FUNCTION "fc_h25_NoRunDG" : VOID
TITLE =Check, if no diesel running on the foreign busbars
//version!date    !author !change_segm!change_description
//-------+--------+-------+-----------+-------------------------------
// 1.0   !27.04.00!Kahle  ! ---       ! 1st version
// 1.1   !09.05.00!Kahle  ! 2,3       ! corr. program
AUTHOR : Kahle
FAMILY : PMA71_SC
NAME : NoFrgnDG
VERSION : 1.0


VAR_OUTPUT
  OUT_Noforeign_run : BOOL ;	//No diesel on the foreign busbars is running
  OUT_AtOneDG_run : BOOL ;	//At least one diesel is running on busbar
END_VAR
VAR_TEMP
  cfg_own : WORD ;	//configuration of the own busbar (of this shore connection)
  cfg_foreign : WORD ;	//configuration of the foreign busbars
  cfg_act : WORD ;	//actual configuration without shoreconnection, EG
  cnt_foreign : BYTE ;	//loop counter "foreign diesel"
  cnt_own : BYTE ;	//loop counter "own diesel"
  act_DB : WORD ;	//actual datablock ot the receive buffer
  foreignDG_run : BOOL ;	//at least one foreign diesel is running with closed generator breaker
  ownDG_run : BOOL ;	//at least one diesel is running on busbar
END_VAR
BEGIN
NETWORK
TITLE =Determine the configuration of the own busbar

      L     "prm_pma".p_bus_part;
      SLW   4; //convert to pointer *2 (=INT)
      LAR1  ;
      AUF   "prm_pma";
      L     DBW [AR1,P#22.0];
      L     W#16#1FFF;
      UW    ; //without EG, shore conn 1, shore conn 2
      T     #cfg_own; //configuration of the own busbar (of this shore connection)


NETWORK
TITLE =Determine the configuration of the foreign busbars

      L     "MEM".o51_actCfg;
      L     W#16#1FFF;
      UW    ; //configuration of the foreign busbar without EG, shore conn 1, shore conn 2
      L     #cfg_own;
      INVI  ;
      UW    ;
      T     #cfg_foreign;
NETWORK
TITLE =Check if a diesel is running on the foreign busbars

      CLR   ;
      =     #foreignDG_run;
      L     13;
lpfg: T     #cnt_foreign;
      L     #cfg_foreign;
      SRW   ;
      SPZ   nxfg; //no diesel defined ...next one

      L     #cnt_foreign;
      +     108;
      T     #act_DB;

      AUF   DB [#act_DB];
      UN    DBX   38.2; //f_brk_clseG1
      SPB   nxfg; //breaker not closed ...next one

      S     #foreignDG_run; //breaker closed -->set flag

nxfg: L     #cnt_foreign;
      LOOP  lpfg;

NETWORK
TITLE =output parameter

      UN    #foreignDG_run;
      =     #OUT_Noforeign_run;

NETWORK
TITLE =Determine the configuration of the own busbars or common busbar

      L     "MEM".o51_actCfg;
      L     W#16#1FFF;
      UW    ; //configuration of the own busbar without EG, shore conn 1, shore conn 2
      T     #cfg_act;
NETWORK
TITLE =Check if a diesel is running on the own busbars

      CLR   ;
      =     #ownDG_run;
      L     13;
lpow: T     #cnt_own;
      L     #cfg_act;
      SRW   ;
      SPZ   nxow; //no diesel defined ...next one

      L     #cnt_own;
      +     108;
      T     #act_DB;

      AUF   DB [#act_DB];
      UN    DBX   38.2; //f_brk_clseG1
      SPB   nxow; //breaker not closed ...next one

      S     #ownDG_run; //breaker closed -->set flag

nxow: L     #cnt_own;
      LOOP  lpow;

      U     #ownDG_run;
      =     #OUT_AtOneDG_run;
END_FUNCTION


FUNCTION "fc_h22_TotLoad" : VOID
TITLE =calculation of the total power of the actual busbar
AUTHOR : Kahle
FAMILY : PMA71
NAME : MeanValu
VERSION : 1.0


VAR_INPUT
  IN_actCfg : WORD ;	//actual configuration (.0:G1 - .12:G13, .13/.14:S1,S2 , .15:EG)
END_VAR
VAR_OUTPUT
  OUT_total_load : DINT ;	//Total load [kW]
  OUT_No_busbar : INT ;	//Number of generator on busbar
END_VAR
VAR_TEMP
  MPI_cnt : BYTE ;	//MPI received data area loop counter
  MPI_DB : INT ;	//MPI received DB
  load_total : DINT ;	//temporary total load [kW]
  Onbus_No : BYTE ;	//Number of generators on busbar
END_VAR
BEGIN
NETWORK
TITLE =intial.internal variables

      L     0;
      T     #load_total;
      T     #Onbus_No;
NETWORK
TITLE =calculate the mean value of the load signals

      L     14;
lpmv: T     #MPI_cnt;
      L     #IN_actCfg;
      SRW   ;
      SPZ   nxmv; //if generator'x' no defined then ...next one

      L     #MPI_cnt;
      +     108;
      T     #MPI_DB;
      AUF   DB [#MPI_DB];

// check if generator'x' on bus
      U     DBX   38.2;
      SPBN  onbs; //if f_brk_clse' =false then ...next one

//add up the actual load
      L     DBW   42;
      ITD   ;
      L     #load_total;
      +D    ;
      T     #load_total; //a_loadG'x'

//add number of generators on busbar
onbs: U     DBX   38.3;
      SPBN  nxmv; //if f_onbus =false then ...next one
      L     #Onbus_No;
      +     1;
      T     #Onbus_No;

//next generator
nxmv: L     #MPI_cnt;

      LOOP  lpmv;

//output
      L     #load_total;
      T     #OUT_total_load;
      L     #Onbus_No;
      T     #OUT_No_busbar;
END_FUNCTION

FUNCTION_BLOCK "fb_522_addAlarm"
TITLE =Additional shore connection protection function (->FB56)
AUTHOR : Kahle
FAMILY : PMA71_SC
NAME : SC_Alarm
VERSION : 1.0


VAR_INPUT
  in_PrtcEG_sign : DWORD ;	//Protection signals especially emergency diesel
END_VAR
VAR_OUTPUT
  out_Fail_Warn_Curr_I : BOOL ;	//Indication "warning Overcurrent I"
  out_Fail_Warn_Curr_II : BOOL ;	//Indication "warning Overcurrent II"
  out_Fail_Warn_Load_I : BOOL ;	//Indication "warning Load I"
  out_Fail_Warn_Load_II : BOOL ;	//Indication "warning Load II"
END_VAR
VAR_TEMP
  temp_Limit_I1 : BOOL ;	//Generator current, limit 1 exceeded (Standby start)
  temp_Limit_I2 : BOOL ;	//Generator current, limit 2 exceeded (Standby start)
  temp_Limit_I3 : BOOL ;	//Generator current, limit 3 exceeded (Uness. consumers 1)
  temp_Limit_I4 : BOOL ;	//Generator current, limit 4 exceeded (Uness. consumers 2)
  temp_Limit_I5 : BOOL ;	//Generator current, limit 5 exceeded (Uness. consumers 3)
  temp_Limit_I6 : BOOL ;	//Generator current, limit 6 exceeded (Standby start, Uness. consumers 1-3)
  temp_Limit_I7 : BOOL ;	//Generator current, limit 7 exceeded (Generator breaker Off)
  temp_Limit_P1 : BOOL ;	//Generator load, limit 1 exceeded (Standby start)
  temp_Limit_P2 : BOOL ;	//Generator load, limit 2 exceeded (Standby start)
  temp_Limit_P3 : BOOL ;	//Generator load, limit 3 exceeded (Uness. consumers 1)
  temp_Limit_P4 : BOOL ;	//Generator load, limit 4 exceeded (Uness. consumers 2)
  temp_Limit_P5 : BOOL ;	//Generator load, limit 5 exceeded (Uness. consumers 3)
  temp_Limit_P6 : BOOL ;	//Generator load, limit 6 exceeded (Standby start, Uness. consumers 1, 2, 3)
  temp_Limit_P7 : BOOL ;	//Generator load, limit 7 exceeded (Gen. breaker Off)
  temp_Limit_f1 : BOOL ;	//Busbar frequency, limit 1 exceeded (Standby start)
  temp_Limit_f2 : BOOL ;	//Busbar frequency, limit 2 exceeded (Standby start)
  temp_Limit_f3 : BOOL ;	//Busbar frequency, limit 3 exceeded (Uness. consumers 1)
  temp_Limit_f4 : BOOL ;	//Busbar frequency, limit 4 exceeded (Uness. consumers 2)
  temp_Limit_f5 : BOOL ;	//Busbar frequency, limit 5 exceeded (Uness. consumers 3)
  temp_Limit_f6 : BOOL ;	//Busbar frequency, limit 6 exceeded (Standby start, Uness. consumers 1, 2, 3)
  temp_Limit_f7 : BOOL ;	//Busbar frequency, limit 7 exceeded (Gen. breaker Off)
  temp_Limit_f8 : BOOL ;	//Busbar frequency, limit 8 exceeded (Overfrequency alarm)
  temp_Limit_U1 : BOOL ;	//Busbar voltage, limit 1 exceeded (Undervoltage, standby start)
  temp_Limit_U2 : BOOL ;	//Busbar voltage, limit 2 exceeded (Undervoltage, Gen. breaker Off)
  temp_Limit_U3 : BOOL ;	//Busbar voltage, limit 3 exceeded (Overvoltage, standby start)
  temp_Limit_U4 : BOOL ;	//Busbar voltage, limit 4 exceeded (Overvoltage, blocking of voltage controller)
  temp_Limit_P7_undel : BOOL ;	//Generator load, limit 7 exceeded, undelayed (Gen. breaker Off)
  temp_Limit_P7_Warn : BOOL ;	//Generator load, limit 7 exceeded, protection warning
  temp_ShortCircuit : BOOL ;	//Latch for signal "Short circuit"
  temp_Wind_Overtemp : BOOL ;	//Generator winding overtemperature, time delayed
  temp_Standby_ProtWarn : BOOL ;	//Request for standby start (EG: Protection warning)
  temp_Uness1_TransfLBrk : BOOL ;	//Trip command for unessential consumers 1 (EG: Trip of transfer line CB)
  temp_Harb_Feedb_Mode : BOOL ;	//Emergency generator in harbour mode or in power feedback mode
END_VAR
BEGIN
NETWORK
TITLE =Load protection signals into the internal store
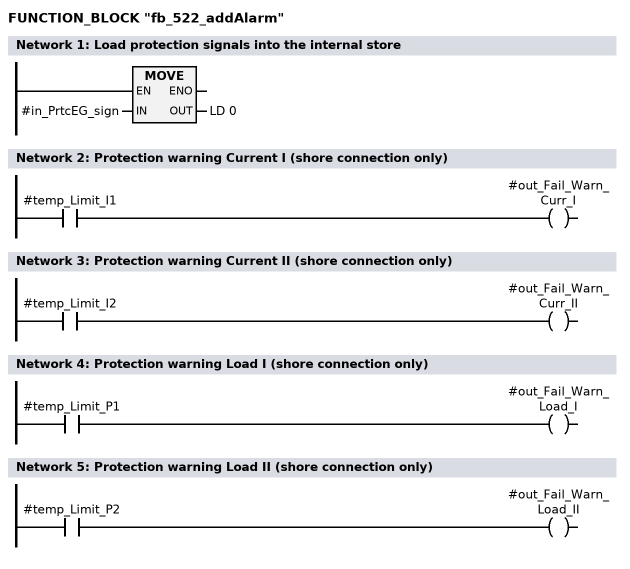
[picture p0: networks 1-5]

      L     #in_PrtcEG_sign;
      T     LD     0; //temp_Limit_I1...
NETWORK
TITLE =Protection warning Current I (shore connection only)

      U     #temp_Limit_I1;
      =     #out_Fail_Warn_Curr_I;
NETWORK
TITLE =Protection warning Current II (shore connection only)

      U     #temp_Limit_I2;
      =     #out_Fail_Warn_Curr_II;
NETWORK
TITLE =Protection warning Load I (shore connection only)

      U     #temp_Limit_P1;
      =     #out_Fail_Warn_Load_I;
NETWORK
TITLE =Protection warning Load II (shore connection only)

      U     #temp_Limit_P2;
      =     #out_Fail_Warn_Load_II;
END_FUNCTION_BLOCK

FUNCTION_BLOCK "fc_522_adjustVolt"
TITLE =Adjusting voltage busbar/ shore connection
//version!date    !author !change_segm!change_description
//-------+--------+-------+-----------+-------------------------------
// 1.0   !01.03.00!Kahle  ! ---       ! 1st version
// 1.1   !18.04.00!Kahle  ! 1(new)    !store signal "adjusting active"
//       !        !       ! 2,3       !signal "#stat_adjustActive" instead of
//       !        !       !           !       "IN_req_adjust"
//       !        !       ! 3         !signal "OUT_adjust" independent from signal
//       !        !       !           !       "#OUT_voltOK_mem
//  1.2  !19.04.00!Kahle  ! 1         !start timer "adjusting voltage"
//       !        !       ! 2         !limit "voltage difference" adjustable
//       !        !       ! 3         !conditions for output "OUT_adjust" are
//       !        !       !           !changed
//  1.3  !09.05.00!Kahle  ! div       !new para: start monit.T
//       !        !       !           !
//       !        !       !           !
//       !        !       !           !
//       !        !       !           !
//       !        !       !           !
//       !        !       !           !
//
AUTHOR : Kahle
FAMILY : PMA71
NAME : AjstVolt
VERSION : 1.3


VAR_INPUT
  IN_strt_adjust : BOOL ;	//start adjusting voltage between busbar and shore connection
  IN_stp_adjust : BOOL ;	//stop adjusting voltage between busbar and shore connection
  IN_strt_wait : BOOL ;	//start waiting time "adjusting voltage"
  IN_bus_L1_L2 : INT ;	//voltage busbar L1/L2
  IN_bus_L3_L1 : INT ;	//voltage busbar L3/L1
  IN_bus_L2_L3 : INT ;	//voltage busbar L2/L3
  IN_shore_L1_L2 : INT ;	//voltage shore connection L1/L2
  IN_shore_L3_L1 : INT ;	//voltage shore connection L3/L1
  IN_shore_L2_L3 : INT ;	//voltage shore connection L2/L3
  IN_Timer_dlyTAdjust : TIMER ;	//Timer "delay time voltage adjusting"
  IN_Timer_MonitAdjust : TIMER ;	//Timer "monitoring voltage adjusting"
  IN_reset : BOOL ;	//Reset failure
END_VAR
VAR_OUTPUT
  OUT_adjust : BOOL ;	//Adjusting voltage
  OUT_failAdjust : BOOL ;	//Failure: Adjusting voltage
END_VAR
VAR_IN_OUT
  OUT_voltOK_mem : BOOL ;	//Voltage between busbar and shore connection ok
END_VAR
VAR
  stat_adjustActive : BOOL ;	//Voltage adjusting is active
  stat_waitTAdjust : BOOL ;	//Waiting time "adjusting" is active
  stat_adjustFail : BOOL ;	//Failure: adjusting voltage
END_VAR
VAR_TEMP
  temp_L1L2unequal : BOOL ;	//voltage L1_L2 between busbar and shore connection is not equal
  temp_L1L3unequal : BOOL ;	//voltage L1_L3 between busbar and shore connection is not equal
  temp_L2L3unequal : BOOL ;	//voltage L2_L3 between busbar and shore connection is not equal
  temp_L1L2equal : BOOL ;	//voltage L1_L2 between busbar and shore connection is equal
  temp_L1L3equal : BOOL ;	//voltage L1_L3 between busbar and shore connection is equal
  temp_L2L3equal : BOOL ;	//voltage L2_L3 between busbar and shore connection is equal
END_VAR
BEGIN
NETWORK
TITLE =Store "voltage adjusting"
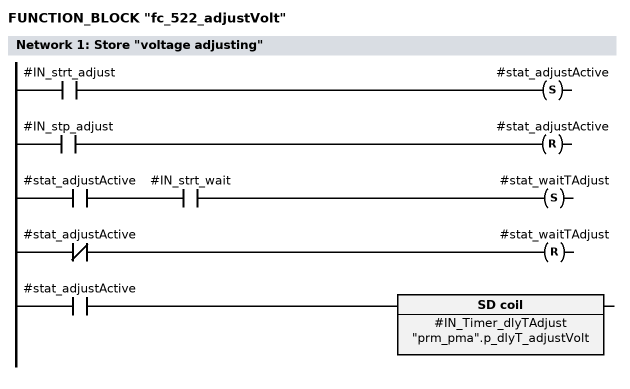
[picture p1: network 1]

      U     #IN_strt_adjust;
      S     #stat_adjustActive;
      U     #IN_stp_adjust;
      R     #stat_adjustActive;

      U     #stat_adjustActive;
      U     #IN_strt_wait;
      S     #stat_waitTAdjust;
      UN    #stat_adjustActive;
      R     #stat_waitTAdjust;

      U     #stat_adjustActive;
      L     "prm_pma".p_dlyT_adjustVolt;
      SE    #IN_Timer_dlyTAdjust;

NETWORK
TITLE =Check voltage between busbar and shore connection and each phas

      UN    #stat_adjustActive;
      SPB   time;

//Check voltage between busbar and shore connection and each phases
      L     #IN_bus_L1_L2;
      L     #IN_shore_L1_L2;
      -I    ;
      PUSH  ;
      SRD   16;
      POP   ;
      SPZ   pos1; //if difference positive ...jump
      NEGI  ;
pos1: L     "I_prtcSR".s_U_DIFF_SET;
      <I    ;
      =     #temp_L1L2equal;
      TAK   ;
      L     "prm_pma".p_allowVoltDiff; //U_DIFF_SET - delta(V)
      -I    ;
      L     "I_prtcSR".s_U_DIFF_SET;
      >I    ;
      =     #temp_L1L2unequal;

      L     #IN_bus_L3_L1;
      L     #IN_shore_L3_L1;
      -I    ;
      PUSH  ;
      SRD   16;
      POP   ;
      SPZ   pos3; //if difference positive ...jump
      NEGI  ;
pos3: L     "I_prtcSR".s_U_DIFF_SET;
      <I    ;
      =     #temp_L1L3equal;
      TAK   ;
      L     "prm_pma".p_allowVoltDiff; //U_DIFF_SET - delta(V)
      -I    ;
      L     "I_prtcSR".s_U_DIFF_SET;
      >I    ;
      =     #temp_L1L3unequal;

      L     #IN_bus_L2_L3;
      L     #IN_shore_L2_L3;
      -I    ;
      PUSH  ;
      SRD   16;
      POP   ;
      SPZ   pos2; //if difference positive ...jump
      NEGI  ;
pos2: L     "I_prtcSR".s_U_DIFF_SET;
      <I    ;
      =     #temp_L2L3equal;
      TAK   ;
      L     "prm_pma".p_allowVoltDiff; //U_DIFF_SET - delta(V)
      -I    ;
      L     "I_prtcSR".s_U_DIFF_SET;
      >I    ;
      =     #temp_L2L3unequal;

      U     #temp_L1L2equal;
      U     #temp_L1L3equal;
      U     #temp_L2L3equal;
      S     #OUT_voltOK_mem;

      O     #temp_L1L2unequal;
      O     #temp_L1L3unequal;
      O     #temp_L2L3unequal;
      R     #OUT_voltOK_mem;


NETWORK
TITLE =Adjusting the voltage between busbar and shore connection
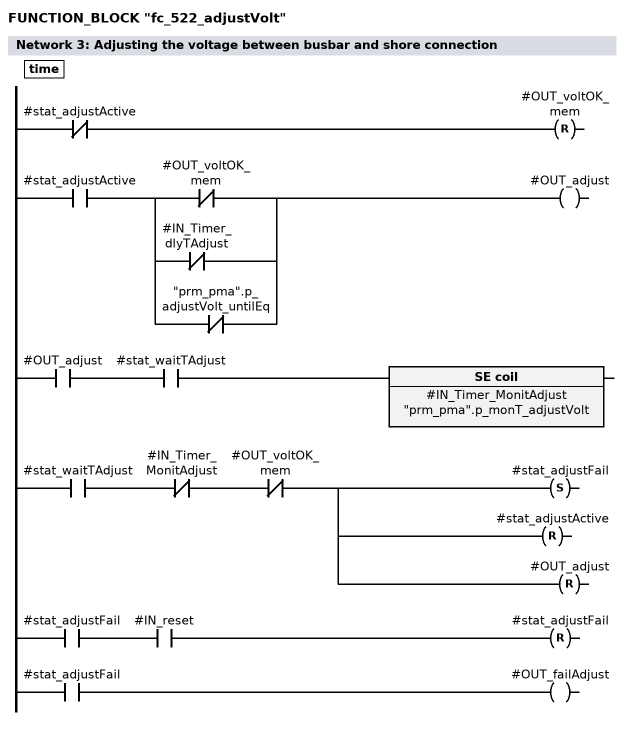
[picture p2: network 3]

time: ON    #stat_adjustActive;
      R     #OUT_voltOK_mem;

      U     #stat_adjustActive;
      U(    ;
      ON    #OUT_voltOK_mem;
      ON    #IN_Timer_dlyTAdjust;
      ON    "prm_pma".p_adjustVolt_untilEq;
      )     ;
      =     #OUT_adjust;

//monitoring time for adjusting voltage
      U     #OUT_adjust;
      U     #stat_waitTAdjust;
      L     "prm_pma".p_monT_adjustVolt;
      SV    #IN_Timer_MonitAdjust;

//monitoring time finished without compensation
      U     #stat_waitTAdjust;
      UN    #IN_Timer_MonitAdjust;
      UN    #OUT_voltOK_mem;
      S     #stat_adjustFail;
      R     #stat_adjustActive;
      R     #OUT_adjust;

      U     #stat_adjustFail;
      U     #IN_reset;
      R     #stat_adjustFail;

      U     #stat_adjustFail;
      =     #OUT_failAdjust;
END_FUNCTION_BLOCK

FUNCTION_BLOCK "fb_522_shoreConn"
TITLE =Shore connection monitoring
//This program controlled the following functions:
//
// - Check the release conditions
// - Lock / release the controller in the generator sets
// - Monitoring of the shutdown criteria
//
//version!date    !author !change_segm!change_description
//-------+--------+-------+-----------+-------------------------------
// 1.0   !26.03.00!Kahle  ! ---       ! 1st version
// 1.1   !18.04.00!Kahle  ! 30        ! Call FB82, new parameter "stop_adjusting"
//       !        !       ! 37        ! add.signal at the para. "IN_simLock"
// 1.2   !09.05.00!Kahle  ! 30        ! parameter "stop_adjusting": shore conn.on
//       !        !       ! 37(new)   ! Adjust voltage whether shore disconn.
//       !        !       ! 37(new    ! Indication "disconn. shore connection"
//       !        !       ! 27        ! signal "shore voltage" connected with
//       !        !       !           ! selector "im-/export"
//       !        !       ! 19(new)   ! Ind "blackout out shore connection"
//       !        !       ! 28        ! external release: new signal "shore on"
//       !        !       !           !                 : "voltage busbar" conn.
//       !        !       !           !                 : with selector
//       !        !       ! 27,28     ! external release: no diesel running on
//       !        !       !           !                   the foreign busbars
//       !        !       ! 42        ! blackout -signal
//       !        !       ! 19,20(new)! blackout monitoring busbar
//       !        !       ! 4,5(new)  ! change selector
//       !        !       ! 26        ! add.alarm "standby start"
//       !        !       ! 29(new)   ! common signal "blackout"
//       !        !       ! 35        ! Start/stop volt.adjust:new commands
//       !        !       ! 36        ! Stop Diesel: signals are changed
//       !        !       ! 38        ! Warn.Stop DG: signals are changed
//       !        !       ! 39        ! Open breaker: signals are changed
//       !        !       ! 40(new)   ! Alarm "DG doesn't stop"
//       !        !       ! 41(new)   ! Signal "absolute value of load signal"
//       !        !       ! 44        ! add signal "selector"
//       !        !       ! 45        ! reset "#stat_indShore_dis" add.signals
//       !        !       ! 46        ! stop adjust.: add.signals
//       !        !       ! 47(new)   ! Alarm "standby start failure"
//       !        !       ! 48        ! reset "#step1_c_brk_off": add.signals
//       !        !       ! 49        ! Alarm "take over load"
//       !        !       ! 50        ! Var.changes "Failure Diesel takeover load"
//       !        !       ! 51        ! Var.changes "Diesel takeover load(import)
//       !        !       ! 52(new)   ! Diesel take over load (mode =export)
//       !        !       ! 53(new)   ! Diesel take over load INDICATION
//       !        !       ! 54        ! Parameter "GB open with red": add.signal
//       !        !       !           ! Parameter "PB GB open": new signal
//       !        !       ! 58        ! Alarm "standby" deleted
//       !        !       ! 59(new)   ! Alarm "standby"
//       !        !       ! 60(new)   ! Alarm "blackout expected"
//       !        !       ! 77        ! Add.signals "blocked"
// 1.3   !20.07.00!Kahle  ! 26,59     ! Alarm'standbyStart" external few sec.only
// 1.4   !14.05.01!Kahle  ! 23        ! Add.ind "OUT_e_I_ov" & "OUT_e_P_ov"
//       !        !       ! 54        ! Add.signals "IN_extShoreBrk_openCmd",
//       !        !       !           ! Add.signals "IN_extBlock"
//
AUTHOR : Kahle
FAMILY : PMA71_SC
NAME : TieMonit
VERSION : 1.4


VAR_INPUT
  IN_selector : BOOL ;	//=0: IMPORT, =1: EXPORT
  IN_cmd_ShoreBrk_on : BOOL ;	//Command shore breaker on
  IN_cmd_ShoreBrk_off : BOOL ;	//Command shore breaker off
  IN_PB_ShoreBrk_off : BOOL ;	//PB shore conn breaker off
  IN_extShoreBrk_openCmd : BOOL ;	//External shore connection open command
  IN_extBlock : BOOL ;	//External blocking is active
  IN_blackout_bus : BOOL ;	//Blackout is detected on the busbar
  IN_VoltAvail_bus : BOOL ;	//Voltage available on the busbar
  IN_blackout_shore : BOOL ;	//Blackout is detected on the shore connection
  IN_shoreVoltAvail : BOOL ;	//Voltage on the shore connection is available
  IN_shortCircuit_otherG : BOOL ;	//At least one generator set has a short circuit detected
  IN_atLeastOneAuto : BOOL ;	//At least one generator set is in automatic
  IN_shortCircuit_ext : BOOL ;	//External device has a short circuit dedected
  IN_atLeastOneAutoOnbus : BOOL ;	//At least one generator set on bus in automatic
  IN_atLeastOneBrkClse : BOOL ;	//At least one generator set is on the busbar
  IN_atLeastShoreOn : BOOL ;	//At least one shore connection is on
  IN_atLeastDGrun : BOOL ;	//At least ond generator set is running
  IN_actCfg : WORD ;	//Actual configuration
  IN_GEN_I_L1 : INT ;	//GENOP71: I_L1
  IN_GEN_I_L2 : INT ;	//GENOP71: I_L2
  IN_GEN_I_L3 : INT ;	//GENOP71: I_L3
  IN_LOAD : INT ;	//GENOP71: active power [in kW]
  IN_BUS_f : INT ;	//GENOP71: f_bus
  IN_GEN_f : INT ;	//GENOP71: f_gen
  IN_BUS_U_L1L2 : INT ;	//GENOP71: U_L1L2_bus
  IN_BUS_U_L2L3 : INT ;	//GENOP71: U_L2L3_bus
  IN_BUS_U_L1L3 : INT ;	//GENOP71: U_L1L3_bus
  IN_GEN_U_L1L2 : INT ;	//GENOP71: U_L1L2_gen
  IN_GEN_U_L2L3 : INT ;	//GENOP71: U_L2L3_gen
  IN_GEN_U_L1L3 : INT ;	//GENOP71: U_L1L3_gen
  IN_I_SC_GW1 : BOOL ;	//GENOP71: I_SC_GW1
  IN_I_GW1VER : BOOL ;	//GENOP71: I_GW1VER
  IN_I_GW2VER : BOOL ;	//GENOP71: I_GW2VER
  IN_I_GW3VER : BOOL ;	//GENOP71: I_GW3VER
  IN_I_GW4VER : BOOL ;	//GENOP71: I_GW4VER
  IN_P_GW1VER : BOOL ;	//GENOP71: P_GW1VER
  IN_simLock_blc : BOOL ;	//Simultaneous lock is blocked
  IN_simLock_err : BOOL ;	//Simultaneous lock failure
  IN_simLockRel : BOOL ;	//Simultaneous lock release
  IN_shoreBrk_trip : BOOL ;	//Shore breaker tripped
  IN_brk_ready : BOOL ;	//Breaker is ready for closing
  IN_brk_normPos : BOOL ;	//Breaker is in norm position
  IN_brk_testPos : BOOL ;	//Breaker is in test position
  IN_brk_on : BOOL ;	//Feedback: breaker is on
  IN_brk_off : BOOL ;	//Feedback: breaker is off
  IN_f_cmdBrkOn : BOOL ;	//Genop Feedback: command breaker on
  IN_reset : BOOL ;	//Reset command
  IN_resetBlock : BOOL ;	//Reset blocking
  IN_pressCnfrm : BOOL ;	//indication: press confirmation
  IN_mode : BYTE ;	//Actual mode (x.0:local, x.1:semiOP, x.2:autoOP, x.3:semi, x.4:auto, x.5:test)
  IN_TimerStdbyStrt : TIMER ;	//Timer startpulse "standby start"
  IN_TimerStpGenSet : TIMER ;	//Timer monitoring generator set stop
  IN_TimerStpPulse : TIMER ;	//Timer stoppulse "diesel"
  IN_TimerMonStdbyStrt : TIMER ;	//Timer monitoring generator set start
  IN_TimerTakeLoad : TIMER ;	//Timer monitoring take over load generator set
END_VAR
VAR_OUTPUT
  OUT_SynchrActive : BOOL ;	//Command: switch up/down
  OUT_c_LckCtrl : BOOL ;	//Command: controller lock
  OUT_c_simLock : BOOL ;	//Command: simultanoeus lock active
  OUT_c_brkON : BOOL ;	//GENOP Command: breaker on
  OUT_c_brkOFF : BOOL ;	//GENOP Command: breaker off
  OUT_c_synRel : BOOL ;	//GENOP Command: synchronizing release
  OUT_c_reqStrt : BOOL ;	//Command: request standby start
  OUT_c_reqStp : BOOL ;	//Command: request stop generator set
  OUT_c_adjustVolt : BOOL ;	//Command: Adjusting voltage
  OUT_c_takeoverLoad : BOOL ;	//Command: take over load
  OUT_c_shortCirc : BOOL ;	//Command: short circuit, open breaker
  OUT_i_blocked : BOOL ;	//Indication: shore connection is blocked
  OUT_i_disconn : BOOL ;	//Indication: disconning shore connection
  OUT_stdbyNo_1st : BYTE ;	//Number of the actual standby generator
  OUT_e_busbar_monit : BOOL ;	//Failure: busbar monitoring
  OUT_e_shore_monit : BOOL ;	//Failure: shore connection monitoring
  OUT_e_I_monit : BOOL ;	//Failure: current monitoring
  OUT_e_I : BOOL ;	//Failure: CB tripped by overcurrent
  OUT_e_revP : BOOL ;	//Failure: reverse power (active in "export" mode)
  OUT_e_I_ov : BOOL ;	//Failure: overcurrent 1
  OUT_e_P_ov : BOOL ;	//Failure: overload 1
  OUT_e_f1 : BOOL ;	//Failure: underfrequency 1
  OUT_e_f2 : BOOL ;	//Failure: underfrequency 2
  OUT_e_f3 : BOOL ;	//Failure: underfrequency 3
  OUT_e_f4 : BOOL ;	//Failure: overfrequency
  OUT_e_U1 : BOOL ;	//Failure: undervoltage 1
  OUT_e_U2 : BOOL ;	//Failure: undervoltage 2
  OUT_e_U3 : BOOL ;	//Failure: undervoltage 3
  OUT_e_U4 : BOOL ;	//Failure: overvoltage
  OUT_e_I_sc : BOOL ;	//Failure: short circuit
  OUT_e_sc_other : BOOL ;	//Failure: short circuit at other generator set
  OUT_e_I1 : BOOL ;	//Failure: overcurrent I
  OUT_e_I2 : BOOL ;	//Failure: overcurrent II
  OUT_e_P1 : BOOL ;	//Failure: overload I
  OUT_e_P2 : BOOL ;	//Failure: overload II
  OUT_e_black : BOOL ;	//Failure: blackout
  OUT_e_brkRdy : BOOL ;	//Failure: breaker ready
  OUT_e_brkOn : BOOL ;	//Failure: breaker on
  OUT_e_brkOff : BOOL ;	//Failure: breaker off
  OUT_e_brkOnOff : BOOL ;	//Failure: breaker feedbak plausibility
  OUT_e_brkTrip : BOOL ;	//Failure: breaker tripped
  OUT_e_brkTripExt : BOOL ;	//Failure: shore connection breaker tripped extern
  OUT_e_synTime : BOOL ;	//Failure: synchronization time exceeded
  OUT_e_StdbyStart : BOOL ;	//Failure: standby start
  OUT_e_loadTooHigh : BOOL ;	//Failure: Power consumption is too high
  OUT_e_adjustVolt : BOOL ;	//Failure: Adjusting voltage
  OUT_e_warnBlackout : BOOL ;	//Warning: Danger of blackout because of no generator set in automatic
  OUT_e_alarmBlackout : BOOL ;	//Alarm: Danger of blackout because of no generator set in automatic
  OUT_e_stpDieselMan : BOOL ;	//Alarm: Stop diesel manually in case of starting shore connection
  OUT_e_noStpDiesel : BOOL ;	//Alarm: No shore conn in case of no DG stop
  OUT_e_standByStart : BOOL ;	//Alarm: Start standby diesel
  OUT_e_takeOverLoad : BOOL ;	//Alarm: Take over load
  OUT_w_takeOverLoad : BOOL ;	//Warning: Take over load manually
  OUT_ind_ready : BYTE ;	//indication: criteria for breaker ready
  OUT_ind_line1_stat : INT ;	//status indication -line 1-
  out_ind_line2_var : INT ;	//status indication -line 2-
END_VAR
VAR
  Gen_Protect : "fb_511_GenProtect";
  Gen_Breaker : "fb_57_clseopnBrk";
  Add_Warning : "fb_522_addAlarm";
  BlockShoreCnn : BOOL ;	//Shore connection breaker is blocked
  BothSideBlackout : BOOL ;	//Blackout on the entire busbar
  BrkRdyClse : BOOL ;	//Breaker is ready for closing
  Pulse_brk_on : BOOL ;	//Pulse "breaker on"
  step1_c_brk_off : BOOL ;	//Command store "breaker off" -step 1-
  step2_c_brk_off : BOOL ;	//Command store "breaker off" -step 2-
  stat_relSimLock : BOOL ;	//Release simultaneous lock after voltage adjusting
  stat_relClseGenBrk : BOOL ;	//Release close generator breaker
  stat_indShore_dis : BOOL ;	//Disconnecting shore connection is active
  stat_c_shore_on : BOOL ;	//Memory command shore connection on
  stat_negP_TimerStpDG : BOOL ;	//Negative pulse timer "stop diesel"
  stat_failStandBy : BOOL ;	//Failure start standby diesel
  stat_failTakeOver : BOOL ;	//Failure take over load
  stat_failBlackout_SC : BOOL ;	//Failure Blackout shore connection
  stat_selector_imp : BOOL ;	//Memo selector =import
  stat_selector_exp : BOOL ;	//Memo selector =export
  Breaker_control : "fb_57_clseopnBrk";	//Breaker control (close, open, monitoring)
  AdjustVolt_conn : "fc_522_adjustVolt";	//Adjusting voltage whether the shore connection will be connected
  AdjustVolt_disconn : "fc_522_adjustVolt";	//Adjusting voltage whether the shore connection will be disconnected
END_VAR
VAR_TEMP
  temp_OM_Local : BOOL ;	//Active operation mode: Local
  temp_OM_Semi_OP : BOOL ;	//Active operation mode: Semi automatic OP
  temp_OM_Auto_OP : BOOL ;	//Active operation mode: Automatic OP
  temp_OM_Semi_MMI : BOOL ;	//Active operation mode: Semi automatic MMI
  temp_OM_Auto_MMI : BOOL ;	//Active operation mode: Automatic MMI
  temp_OM_Test : BOOL ;	//Active operation mode: Test (EG only)
  temp_Reserve_006 : BOOL ;	//Reserved (Transfer Byte --> Bit)
  temp_Reserve_007 : BOOL ;	//Reserved (Transfer Byte --> Bit)
  temp_ext_release : BOOL ;	//external releases
  temp_shoreBus_on : BOOL ;	//shore connection active at the configuration 1
  temp_shoreTrs_on : BOOL ;	//shore connection active at the configuration 2
  temp_TieOffBlack : BOOL ;	//On side blackout: tie breaker off
  temp_TieOffNoGen : BOOL ;	//Number of allowed generator exceeded: tie breaker off
  temp_req_StdbyStrt : BOOL ;	//Request start standby generator set
  temp_VoltAvailBusPrtct : BOOL ;	//Busbar voltage available
  temp_VoltAvailShorePrtct : BOOL ;	//Shore connection voltage available
  temp_Brk_off : BOOL ;	//Command: breaker off
  temp_block : BOOL ;	//Blocking own breaker
  temp_Auto : BOOL ;	//mode =automatic OP or automatic MMI
  temp_c_brkOff : BOOL ;	//command: breaker off
  temp_c_brkLoadRed : BOOL ;	//command: shore connection breaker off with load reduction
  temp_tieBrk_ready : BOOL ;	//tie breaker ready
  var26 : BOOL ;
  var27 : BOOL ;
  temp_VoltAvailBus : BOOL ;	//voltage busbar available
  temp_VoltAvailShore : BOOL ;	//voltage shore connection available
  temp_blocking : BOOL ;	//Shore connection is blocked
  temp_LoadTooHigh : BOOL ;	//Total load is too high
  temp_Semi : BOOL ;	//Active operation mode: Semi automatic
  temp_normTestPos : BOOL ;	//Breaker in norm or test position
  temp_readyClose : BOOL ;	//Breaker is ready for closing
  temp_brkOff_noLoad : BOOL ;	//Breaker off, load less then minimum
  temp_GEN_I_L1 : INT ;	//Generator current L1 (in 100.00% of nominal value)
  temp_GEN_I_L2 : INT ;	//Generator current L1 (in 100.00% of nominal value)
  temp_GEN_I_L3 : INT ;	//Generator current L1 (in 100.00% of nominal value)
  temp_BUS_f : INT ;	//Bus bar frequency (in 100.00% of nominal value)
  temp_GEN_f : INT ;	//Generator frequency (in 100.00% of nominal value)
  temp_BUS_U_L1L2 : INT ;	//Bus bar voltage L1/L2 (in 100.00% of nominal value)
  temp_BUS_U_L2L3 : INT ;	//Bus bar voltage L2/L3 (in 100.00% of nominal value)
  temp_GEN_P_SUM : INT ;	//Generator active load (in 100.00% of nominal value)
  temp_Operat_Status : INT ;	//status indication for OP7
  temp_BUS_U_L3L1 : INT ;	//Bus bar voltage L3/L1 (in 100.00% of nominal value)
  temp_GEN_U_L1L2 : INT ;	//Generator voltage L1/L2 (in 100.00% of nominal value)
  temp_GEN_U_L2L3 : INT ;	//Generator voltage L2/L3 (in 100.00% of nominal value)
  temp_GEN_U_L3L1 : INT ;	//Generator voltage L3/L1 (in 100.00% of nominal value)
  temp_GenNo_onbus : INT ;	//Number of generator which are on busbar
  temp_CfgBusbar : INT ;	//Actual configration busbar
  temp_CfgTrans : INT ;	//Actual configuration transferline
  temp_Indication2_FB51 : INT ;	//Indication number, line 2, from FB51
  temp_totalLoad : DINT ;	//total load of the actual configuration
  temp_No_busbar : INT ;	//Number of generator in automatic on busbar
  temp_addAlarm : DWORD ;	//Additional shore connection warnings
  temp_c_adjustV_conn : BOOL ;	//command "adjusting voltage" in case connecting to shore
  temp_c_adjustV_disconn : BOOL ;	//command "adjusting voltage" in case disconnecting from shore
  temp_e_adjustV_conn : BOOL ;	//failure "adjusting voltage" in case connecting to shore
  temp_e_adjustV_disconn : BOOL ;	//failure "adjusting voltage" in case disconnecting from shore
  temp_e_blackout : BOOL ;	//failure "blackout shore connection"
  temp_noForeignRun : BOOL ;	//No running diesel on foreign busbars
  temp_atOneDG_run : BOOL ;	//At least one diesel is running on busbar
  temp_blackBus : BOOL ;	//blackout on the busbar
  temp_e_alarmBlack_I : BOOL ;	//Alarm: Blackout expected
  temp_e_alarmBlack_II : BOOL ;	//Alarm: Blackout expected
  temp_blackout : BOOL ;	//blackout
  temp_e_standby_ext : BOOL ;	//Alarm: standby start external
  temp_e_standby_int : BOOL ;	//Alarm: standby start internal
  temp_selec_chgToExp : BOOL ;	//Selector change to export
  temp_selec_chgToImp : BOOL ;	//Selector change to import
  temp_reset_actProcess : BOOL ;	//Reset actual process
  temp_open_withoutRed : BOOL ;	//Open shore connection without load reduction
  temp_GEN_U_Max : INT ;	//Mains (generator) voltage, highest value (phase L1/L2, L2/L3, L3/L1)
END_VAR
BEGIN
NETWORK
TITLE =GENERAL -Move operation mode (Transfer Byte --> Bit)
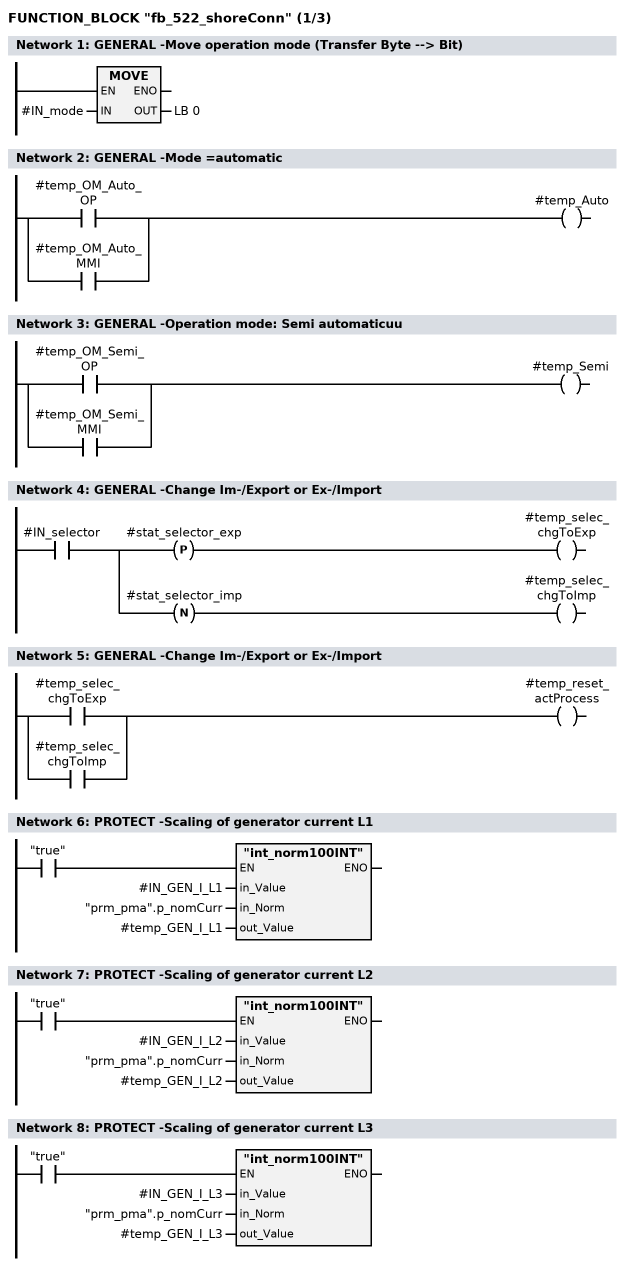
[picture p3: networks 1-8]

      L     #IN_mode;
      T     LB     0;
NETWORK
TITLE =GENERAL -Mode =automatic

      O     #temp_OM_Auto_OP;
      O     #temp_OM_Auto_MMI;
      =     #temp_Auto;
NETWORK
TITLE =GENERAL -Operation mode: Semi automaticuu

      O     #temp_OM_Semi_OP;
      O     #temp_OM_Semi_MMI;
      =     #temp_Semi;
NETWORK
TITLE =GENERAL -Change Im-/Export or Ex-/Import

      U     #IN_selector;
      =     L     54.0;
      U     L     54.0;
      FP    #stat_selector_exp;
      =     #temp_selec_chgToExp;
      U     L     54.0;
      FN    #stat_selector_imp;
      =     #temp_selec_chgToImp;
NETWORK
TITLE =GENERAL -Change Im-/Export or Ex-/Import

      O     #temp_selec_chgToExp;
      O     #temp_selec_chgToImp;
      =     #temp_reset_actProcess;
NETWORK
TITLE =PROTECT -Scaling of generator current L1

      U     "true";
      SPBNB _001;
      CALL "int_norm100INT" (
           in_Value                 := #IN_GEN_I_L1,
           in_Norm                  := "prm_pma".p_nomCurr,
           out_Value                := #temp_GEN_I_L1);
_001: NOP   0;
NETWORK
TITLE =PROTECT -Scaling of generator current L2

      U     "true";
      SPBNB _002;
      CALL "int_norm100INT" (
           in_Value                 := #IN_GEN_I_L2,
           in_Norm                  := "prm_pma".p_nomCurr,
           out_Value                := #temp_GEN_I_L2);
_002: NOP   0;
NETWORK
TITLE =PROTECT -Scaling of generator current L3

      U     "true";
      SPBNB _003;
      CALL "int_norm100INT" (
           in_Value                 := #IN_GEN_I_L3,
           in_Norm                  := "prm_pma".p_nomCurr,
           out_Value                := #temp_GEN_I_L3);
_003: NOP   0;
NETWORK
TITLE =PROTECT -Scaling of busbar frequency
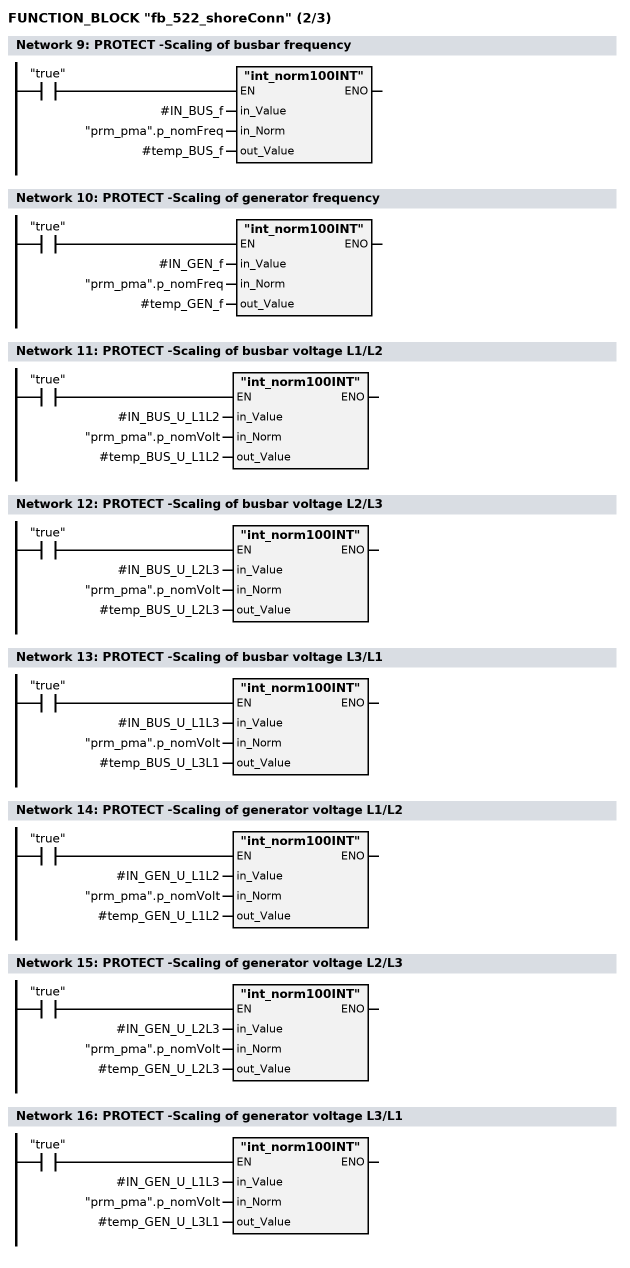
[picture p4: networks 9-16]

      U     "true";
      SPBNB _007;
      CALL "int_norm100INT" (
           in_Value                 := #IN_BUS_f,
           in_Norm                  := "prm_pma".p_nomFreq,
           out_Value                := #temp_BUS_f);
_007: NOP   0;
NETWORK
TITLE =PROTECT -Scaling of generator frequency

      U     "true";
      SPBNB _00b;
      CALL "int_norm100INT" (
           in_Value                 := #IN_GEN_f,
           in_Norm                  := "prm_pma".p_nomFreq,
           out_Value                := #temp_GEN_f);
_00b: NOP   0;
NETWORK
TITLE =PROTECT -Scaling of busbar voltage L1/L2

      U     "true";
      SPBNB _011;
      CALL "int_norm100INT" (
           in_Value                 := #IN_BUS_U_L1L2,
           in_Norm                  := "prm_pma".p_nomVolt,
           out_Value                := #temp_BUS_U_L1L2);
_011: NOP   0;
NETWORK
TITLE =PROTECT -Scaling of busbar voltage L2/L3

      U     "true";
      SPBNB _012;
      CALL "int_norm100INT" (
           in_Value                 := #IN_BUS_U_L2L3,
           in_Norm                  := "prm_pma".p_nomVolt,
           out_Value                := #temp_BUS_U_L2L3);
_012: NOP   0;
NETWORK
TITLE =PROTECT -Scaling of busbar voltage L3/L1

      U     "true";
      SPBNB _013;
      CALL "int_norm100INT" (
           in_Value                 := #IN_BUS_U_L1L3,
           in_Norm                  := "prm_pma".p_nomVolt,
           out_Value                := #temp_BUS_U_L3L1);
_013: NOP   0;
NETWORK
TITLE =PROTECT -Scaling of generator voltage L1/L2

      U     "true";
      SPBNB _017;
      CALL "int_norm100INT" (
           in_Value                 := #IN_GEN_U_L1L2,
           in_Norm                  := "prm_pma".p_nomVolt,
           out_Value                := #temp_GEN_U_L1L2);
_017: NOP   0;
NETWORK
TITLE =PROTECT -Scaling of generator voltage L2/L3

      U     "true";
      SPBNB _01b;
      CALL "int_norm100INT" (
           in_Value                 := #IN_GEN_U_L2L3,
           in_Norm                  := "prm_pma".p_nomVolt,
           out_Value                := #temp_GEN_U_L2L3);
_01b: NOP   0;
NETWORK
TITLE =PROTECT -Scaling of generator voltage L3/L1

      U     "true";
      SPBNB _01c;
      CALL "int_norm100INT" (
           in_Value                 := #IN_GEN_U_L1L3,
           in_Norm                  := "prm_pma".p_nomVolt,
           out_Value                := #temp_GEN_U_L3L1);
_01c: NOP   0;
NETWORK
TITLE =PROTECT -Scaling of generator active load
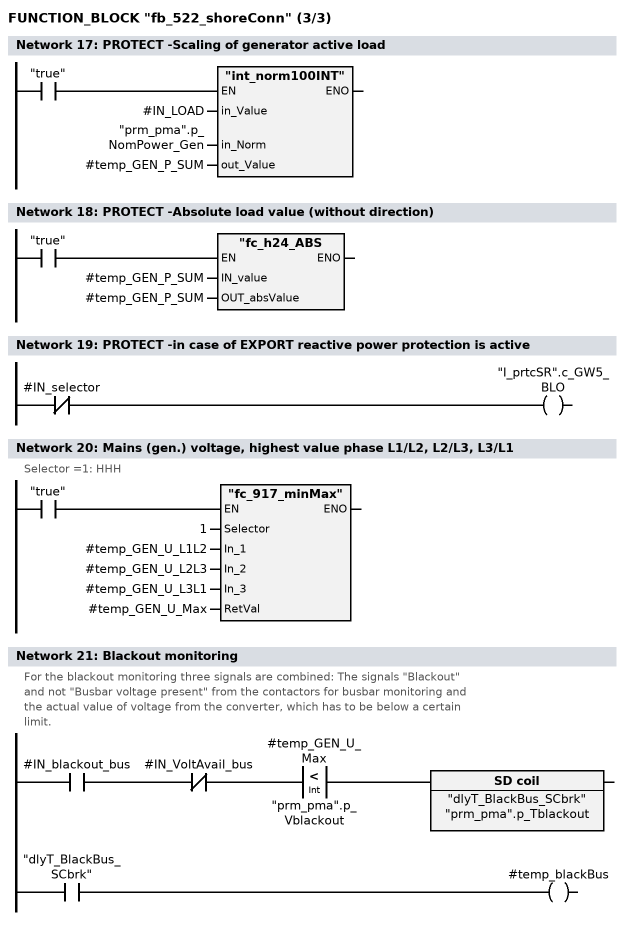
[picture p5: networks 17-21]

      U     "true";
      SPBNB _01d;
      CALL "int_norm100INT" (
           in_Value                 := #IN_LOAD,
           in_Norm                  := "prm_pma".p_NomPower_Gen,
           out_Value                := #temp_GEN_P_SUM);
_01d: NOP   0;
NETWORK
TITLE =PROTECT -Absolute load value (without direction)

      U     "true";
      SPBNB _01e;
      CALL "fc_h24_ABS(INT)" (
           IN_value                 := #temp_GEN_P_SUM,
           OUT_absValue             := #temp_GEN_P_SUM);
_01e: NOP   0;
NETWORK
TITLE =PROTECT -in case of EXPORT reactive power protection is active

      UN    #IN_selector;
      =     "I_prtcSR".c_GW5_BLO;
NETWORK
TITLE =Mains (gen.) voltage, highest value phase L1/L2, L2/L3, L3/L1
//Selector =1: HHH
      U     "true";
      SPBNB _01f;
      CALL "fc_917_minMax" (
           Selector                 := 1,
           In_1                     := #temp_GEN_U_L1L2,
           In_2                     := #temp_GEN_U_L2L3,
           In_3                     := #temp_GEN_U_L3L1,
           RetVal                   := #temp_GEN_U_Max);
_01f: NOP   0;
NETWORK
TITLE =Blackout monitoring
//For the blackout monitoring three signals are combined: The signals "Blackout"
//and not "Busbar voltage present" from the contactors for busbar monitoring and
//the actual value of voltage from the converter, which has to be below a certain
//limit.
      U     #IN_blackout_bus;
      UN    #IN_VoltAvail_bus;
      U(    ;
      L     #temp_GEN_U_Max;
      L     "prm_pma".p_Vblackout;
      <I    ;
      )     ;
      L     "prm_pma".p_Tblackout;
      SE    "dlyT_BlackBus_SCbrk";
      NOP   0;
      NOP   0;
      NOP   0;
      U     "dlyT_BlackBus_SCbrk";
      =     #temp_blackBus;
NETWORK
TITLE =Indication "Failure busbar/blackout monitoring"
//If both signals "Blackout" and "Busbar voltage present" from the contactors for
//busbar monitoring are present or both are not present, there is a failure in
//the
//busbar monitoring.
      U     #IN_reset;
      R     #OUT_e_busbar_monit;
      U(    ;
      U(    ;
      U     #IN_blackout_bus;
      U     #IN_VoltAvail_bus;
      O     ;
      UN    #IN_blackout_bus;
      UN    #IN_VoltAvail_bus;
      )     ;
      L     "prm_pma".p_TFBusbar;
      SE    "dlyT_BusbarFail_SCbrk";
      NOP   0;
      NOP   0;
      NOP   0;
      U     "dlyT_BusbarFail_SCbrk";
      )     ;
      S     #OUT_e_busbar_monit;
      NOP   0;
NETWORK
TITLE =PROTECT -Generator protection (FB56)
//In this case: Generator means busbar, busbar means transferline!
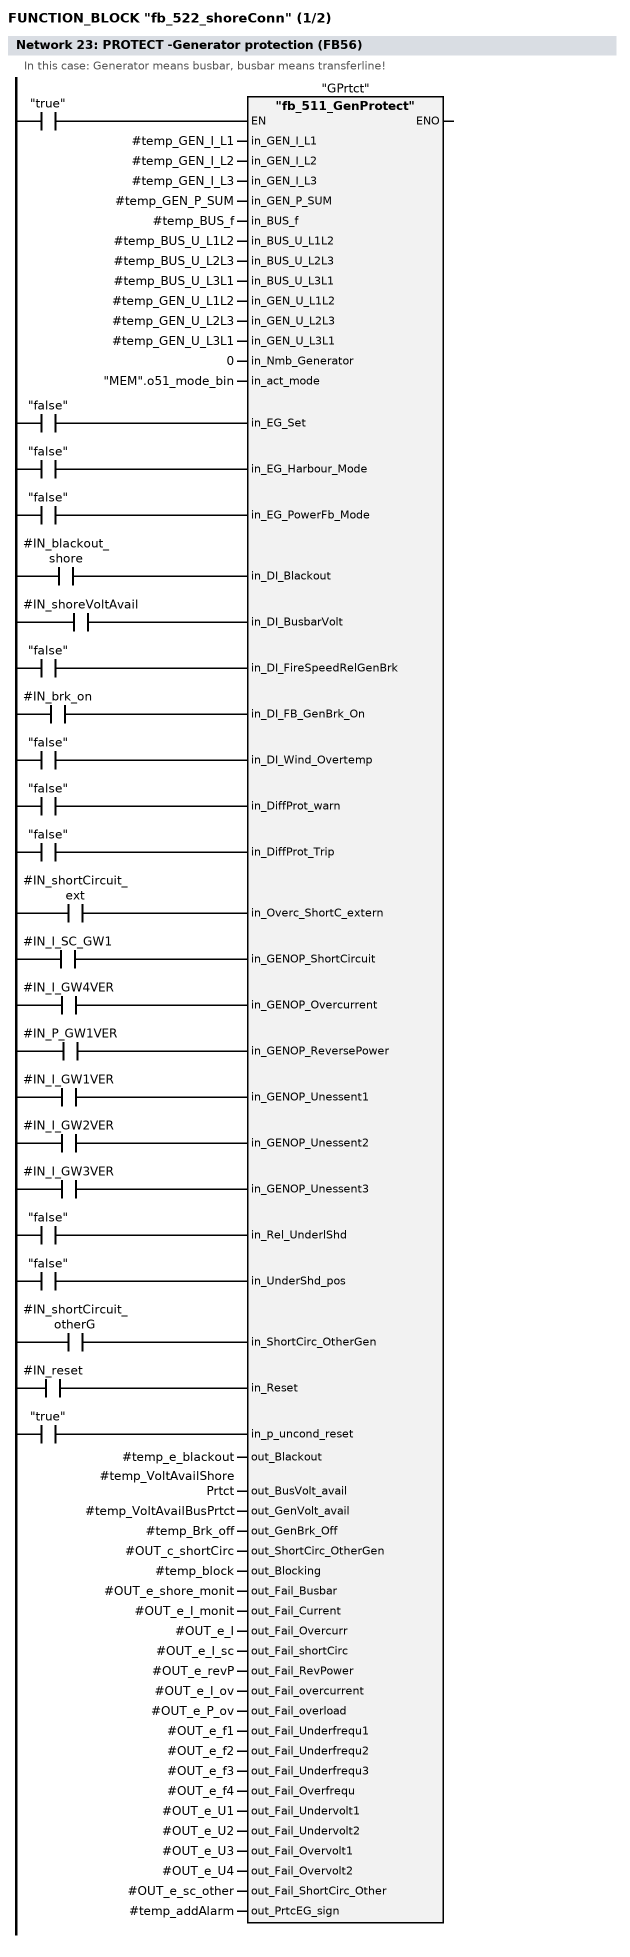
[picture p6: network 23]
      U     "false";
      =     L     54.0;
      BLD   103;
      U     "false";
      =     L     54.1;
      BLD   103;
      U     "false";
      =     L     54.2;
      BLD   103;
      U     #IN_blackout_shore;
      =     L     54.3;
      BLD   103;
      U     #IN_shoreVoltAvail;
      =     L     54.4;
      BLD   103;
      U     "false";
      =     L     54.5;
      BLD   103;
      U     #IN_brk_on;
      =     L     54.6;
      BLD   103;
      U     "false";
      =     L     54.7;
      BLD   103;
      U     "false";
      =     L     55.0;
      BLD   103;
      U     "false";
      =     L     55.1;
      BLD   103;
      U     #IN_shortCircuit_ext;
      =     L     55.2;
      BLD   103;
      U     #IN_I_SC_GW1;
      =     L     55.3;
      BLD   103;
      U     #IN_I_GW4VER;
      =     L     55.4;
      BLD   103;
      U     #IN_P_GW1VER;
      =     L     55.5;
      BLD   103;
      U     #IN_I_GW1VER;
      =     L     55.6;
      BLD   103;
      U     #IN_I_GW2VER;
      =     L     55.7;
      BLD   103;
      U     #IN_I_GW3VER;
      =     L     56.0;
      BLD   103;
      U     "false";
      =     L     56.1;
      BLD   103;
      U     "false";
      =     L     56.2;
      BLD   103;
      U     #IN_shortCircuit_otherG;
      =     L     56.3;
      BLD   103;
      U     #IN_reset;
      =     L     56.4;
      BLD   103;
      U     "true";
      =     L     56.5;
      BLD   103;
      U     "true";
      SPBNB _024;
      CALL "fb_511_GenProtect" , "GPrtct" (
           in_GEN_I_L1              := #temp_GEN_I_L1,
           in_GEN_I_L2              := #temp_GEN_I_L2,
           in_GEN_I_L3              := #temp_GEN_I_L3,
           in_GEN_P_SUM             := #temp_GEN_P_SUM,
           in_BUS_f                 := #temp_BUS_f,
           in_BUS_U_L1L2            := #temp_BUS_U_L1L2,
           in_BUS_U_L2L3            := #temp_BUS_U_L2L3,
           in_BUS_U_L3L1            := #temp_BUS_U_L3L1,
           in_GEN_U_L1L2            := #temp_GEN_U_L1L2,
           in_GEN_U_L2L3            := #temp_GEN_U_L2L3,
           in_GEN_U_L3L1            := #temp_GEN_U_L3L1,
           in_Nmb_Generator         := 0,
           in_act_mode              := "MEM".o51_mode_bin,
           in_EG_Set                := L     54.0,
           in_EG_Harbour_Mode       := L     54.1,
           in_EG_PowerFb_Mode       := L     54.2,
           in_DI_Blackout           := L     54.3,
           in_DI_BusbarVolt         := L     54.4,
           in_DI_FireSpeedRelGenBrk := L     54.5,
           in_DI_FB_GenBrk_On       := L     54.6,
           in_DI_Wind_Overtemp      := L     54.7,
           in_DiffProt_warn         := L     55.0,
           in_DiffProt_Trip         := L     55.1,
           in_Overc_ShortC_extern   := L     55.2,
           in_GENOP_ShortCircuit    := L     55.3,
           in_GENOP_Overcurrent     := L     55.4,
           in_GENOP_ReversePower    := L     55.5,
           in_GENOP_Unessent1       := L     55.6,
           in_GENOP_Unessent2       := L     55.7,
           in_GENOP_Unessent3       := L     56.0,
           in_Rel_UnderlShd         := L     56.1,
           in_UnderShd_pos          := L     56.2,
           in_ShortCirc_OtherGen    := L     56.3,
           in_Reset                 := L     56.4,
           in_p_uncond_reset        := L     56.5,
           out_Blackout             := #temp_e_blackout,
           out_BusVolt_avail        := #temp_VoltAvailShorePrtct,
           out_GenVolt_avail        := #temp_VoltAvailBusPrtct,
           out_GenBrk_Off           := #temp_Brk_off,
           out_ShortCirc_OtherGen   := #OUT_c_shortCirc,
           out_Blocking             := #temp_block,
           out_Fail_Busbar          := #OUT_e_shore_monit,
           out_Fail_Current         := #OUT_e_I_monit,
           out_Fail_Overcurr        := #OUT_e_I,
           out_Fail_shortCirc       := #OUT_e_I_sc,
           out_Fail_RevPower        := #OUT_e_revP,
           out_Fail_overcurrent     := #OUT_e_I_ov,
           out_Fail_overload        := #OUT_e_P_ov,
           out_Fail_Underfrequ1     := #OUT_e_f1,
           out_Fail_Underfrequ2     := #OUT_e_f2,
           out_Fail_Underfrequ3     := #OUT_e_f3,
           out_Fail_Overfrequ       := #OUT_e_f4,
           out_Fail_Undervolt1      := #OUT_e_U1,
           out_Fail_Undervolt2      := #OUT_e_U2,
           out_Fail_Overvolt1       := #OUT_e_U3,
           out_Fail_Overvolt2       := #OUT_e_U4,
           out_Fail_ShortCirc_Other := #OUT_e_sc_other,
           out_PrtcEG_sign          := #temp_addAlarm);
_024: NOP   0;
NETWORK
TITLE =PROTECT -Indication "no shore connection voltage"
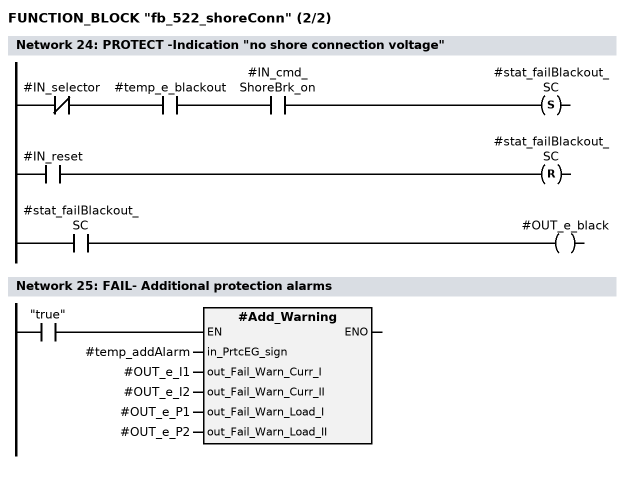
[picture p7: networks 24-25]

      UN    #IN_selector;
      U     #temp_e_blackout;
      U     #IN_cmd_ShoreBrk_on;
      S     #stat_failBlackout_SC;
      U     #IN_reset;
      R     #stat_failBlackout_SC;
      U     #stat_failBlackout_SC;
      =     #OUT_e_black;
NETWORK
TITLE =FAIL- Additional protection alarms

      U     "true";
      SPBNB _025;
      CALL #Add_Warning (
           in_PrtcEG_sign           := #temp_addAlarm,
           out_Fail_Warn_Curr_I     := #OUT_e_I1,
           out_Fail_Warn_Curr_II    := #OUT_e_I2,
           out_Fail_Warn_Load_I     := #OUT_e_P1,
           out_Fail_Warn_Load_II    := #OUT_e_P2);
_025: NOP   0;
NETWORK
TITLE =FAIL- Standby start external shore conn.breaker tripped only

      UN    #IN_selector;
      U     #IN_brk_on;
      U     #IN_shoreBrk_trip;
      =     L     54.0;
      U     L     54.0;
      BLD   102;
      =     #temp_req_StdbyStrt;
      O     L     54.0;
      O     #IN_shoreBrk_trip;
      =     #OUT_e_brkTripExt;
NETWORK
TITLE =PRECON -Determine the actual power consumption
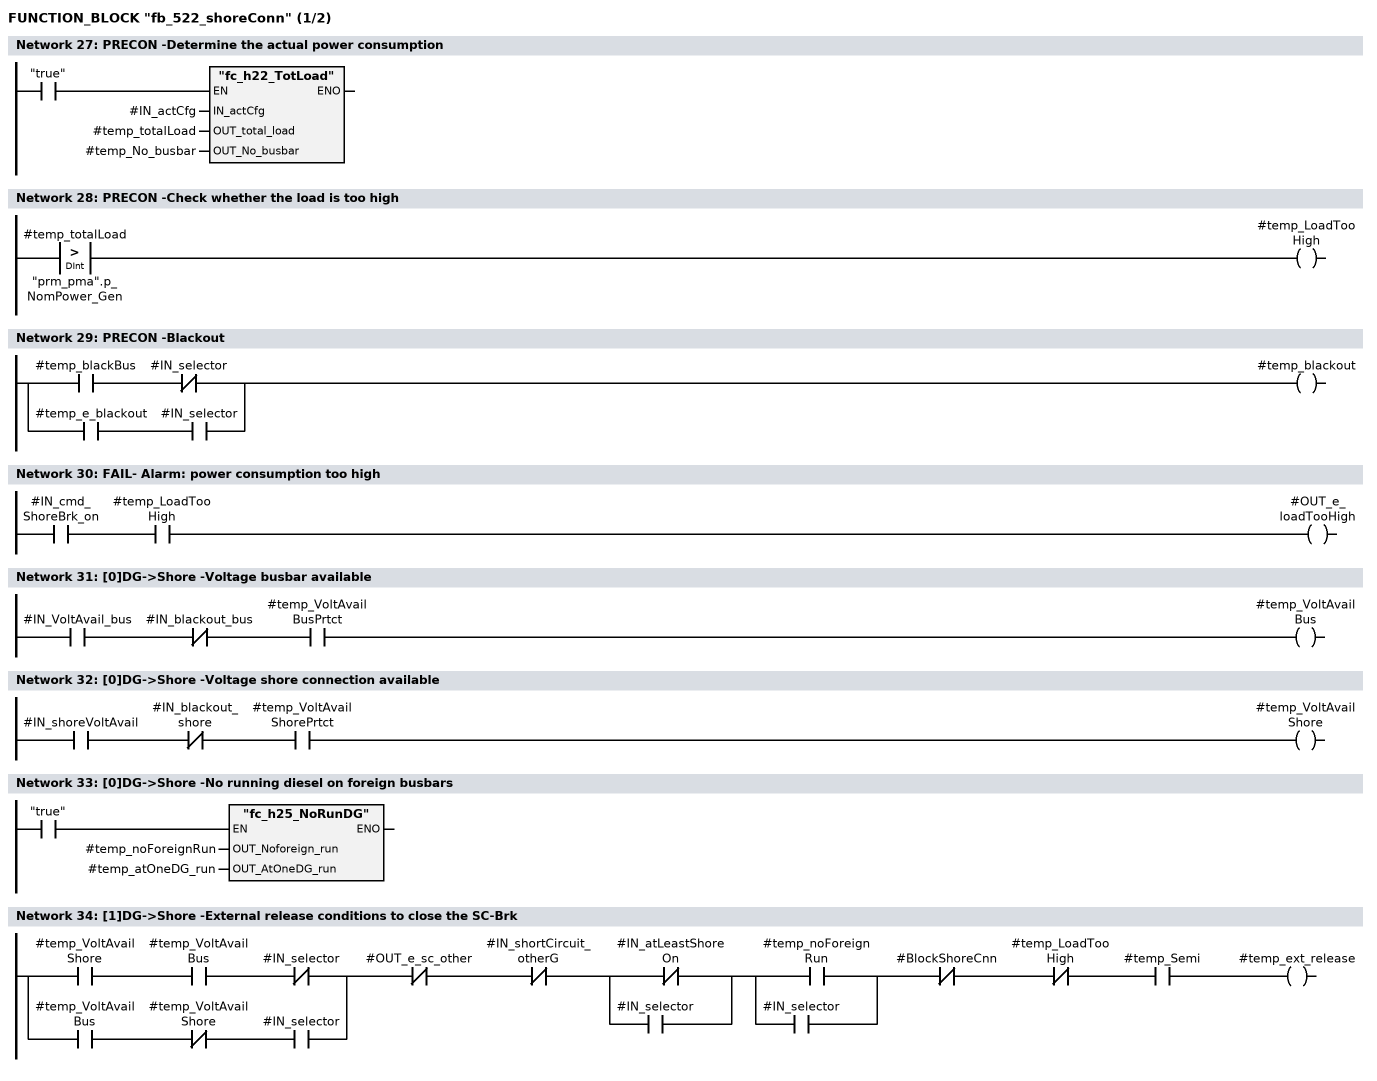
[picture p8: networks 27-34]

      U     "true";
      SPBNB _026;
      CALL "fc_h22_TotLoad" (
           IN_actCfg                := #IN_actCfg,
           OUT_total_load           := #temp_totalLoad,
           OUT_No_busbar            := #temp_No_busbar);
_026: NOP   0;
NETWORK
TITLE =PRECON -Check whether the load is too high

      L     #temp_totalLoad;
      L     "prm_pma".p_NomPower_Gen;
      >D    ;
      =     #temp_LoadTooHigh;

NETWORK
TITLE =PRECON -Blackout

      U     #temp_blackBus;
      UN    #IN_selector;
      O     ;
      U     #temp_e_blackout;
      U     #IN_selector;
      =     #temp_blackout;
NETWORK
TITLE =FAIL- Alarm: power consumption too high

      U     #IN_cmd_ShoreBrk_on;
      U     #temp_LoadTooHigh;
      =     #OUT_e_loadTooHigh;
NETWORK
TITLE =[0]DG->Shore -Voltage busbar available

      U     #IN_VoltAvail_bus;
      UN    #IN_blackout_bus;
      U     #temp_VoltAvailBusPrtct;
      =     #temp_VoltAvailBus;
NETWORK
TITLE =[0]DG->Shore -Voltage shore connection available

      U     #IN_shoreVoltAvail;
      UN    #IN_blackout_shore;
      U     #temp_VoltAvailShorePrtct;
      =     #temp_VoltAvailShore;
NETWORK
TITLE =[0]DG->Shore -No running diesel on foreign busbars

      U     "true";
      SPBNB _027;
      CALL "fc_h25_NoRunDG" (
           OUT_Noforeign_run        := #temp_noForeignRun,
           OUT_AtOneDG_run          := #temp_atOneDG_run);
_027: NOP   0;
NETWORK
TITLE =[1]DG->Shore -External release conditions to close the SC-Brk

      U(    ;
      U     #temp_VoltAvailShore;
      U     #temp_VoltAvailBus;
      UN    #IN_selector;
      O     ;
      U     #temp_VoltAvailBus;
      UN    #temp_VoltAvailShore;
      U     #IN_selector;
      )     ;
      UN    #OUT_e_sc_other;
      UN    #IN_shortCircuit_otherG;
      U(    ;
      ON    #IN_atLeastShoreOn;
      O     #IN_selector;
      )     ;
      U(    ;
      O     #temp_noForeignRun;
      O     #IN_selector;
      )     ;
      UN    #BlockShoreCnn;
      UN    #temp_LoadTooHigh;
      U     #temp_Semi;
      =     #temp_ext_release;
NETWORK
TITLE =[3]DG->Shore -Adjusting the voltage controller
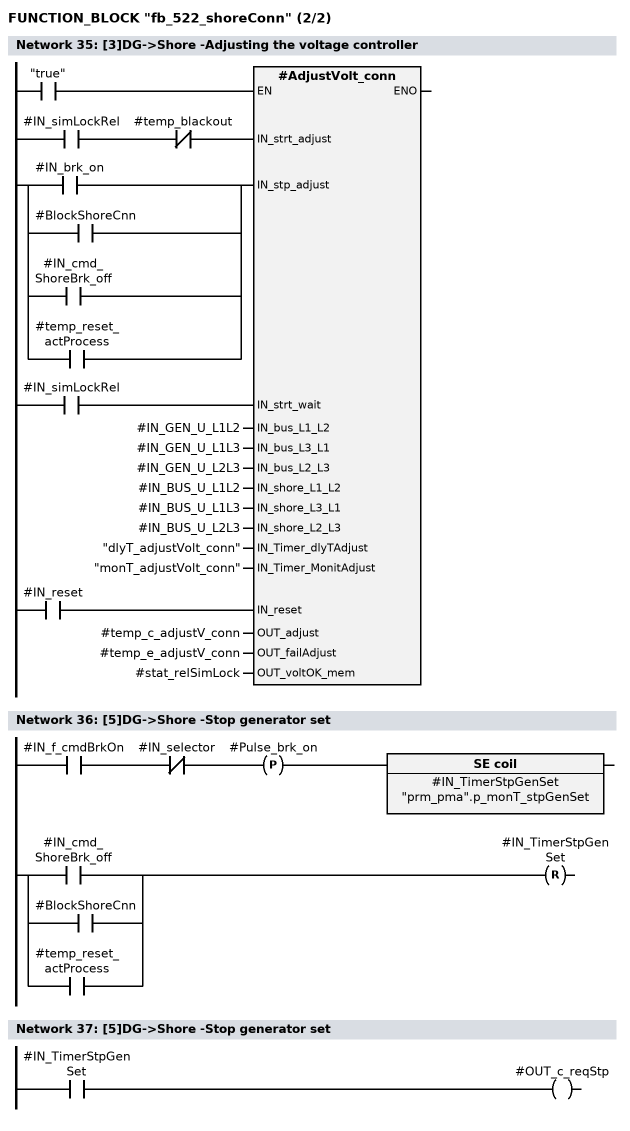
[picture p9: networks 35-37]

      U     #IN_simLockRel;
      UN    #temp_blackout;
      =     L     54.0;
      BLD   103;
      U(    ;
      O     #IN_brk_on;
      O     #BlockShoreCnn;
      O     #IN_cmd_ShoreBrk_off;
      O     #temp_reset_actProcess;
      )     ;
      =     L     54.1;
      BLD   103;
      U     #IN_simLockRel;
      =     L     54.2;
      BLD   103;
      U     #IN_reset;
      =     L     54.3;
      BLD   103;
      U     "true";
      SPBNB _02f;
      CALL #AdjustVolt_conn (
           IN_strt_adjust           := L     54.0,
           IN_stp_adjust            := L     54.1,
           IN_strt_wait             := L     54.2,
           IN_bus_L1_L2             := #IN_GEN_U_L1L2,
           IN_bus_L3_L1             := #IN_GEN_U_L1L3,
           IN_bus_L2_L3             := #IN_GEN_U_L2L3,
           IN_shore_L1_L2           := #IN_BUS_U_L1L2,
           IN_shore_L3_L1           := #IN_BUS_U_L1L3,
           IN_shore_L2_L3           := #IN_BUS_U_L2L3,
           IN_Timer_dlyTAdjust      := "dlyT_adjustVolt_conn",
           IN_Timer_MonitAdjust     := "monT_adjustVolt_conn",
           IN_reset                 := L     54.3,
           OUT_adjust               := #temp_c_adjustV_conn,
           OUT_failAdjust           := #temp_e_adjustV_conn,
           OUT_voltOK_mem           := #stat_relSimLock);
_02f: NOP   0;
NETWORK
TITLE =[5]DG->Shore -Stop generator set

      U     #IN_f_cmdBrkOn;
      UN    #IN_selector;
      FP    #Pulse_brk_on;
      L     "prm_pma".p_monT_stpGenSet;
      SV    #IN_TimerStpGenSet;
      U(    ;
      O     #IN_cmd_ShoreBrk_off;
      O     #BlockShoreCnn;
      O     #temp_reset_actProcess;
      )     ;
      R     #IN_TimerStpGenSet;
      NOP   0;
      NOP   0;
      NOP   0;
NETWORK
TITLE =[5]DG->Shore -Stop generator set

      U     #IN_TimerStpGenSet;
      =     #OUT_c_reqStp;
NETWORK
TITLE =[5]DG->Shore -Alarm: "Stop diesel manually"
//If no diesel in automtic mode set alarm "stop diesel manually"
      UN    "MEM".o515R_f_onbus;
      UN    #temp_blackout;
      UN    #IN_selector;
      U(    ;
      U     #IN_cmd_ShoreBrk_on;
      S     #stat_c_shore_on;
      U(    ;
      O     #IN_simLockRel;
      O     #IN_brk_on;
      O     #BlockShoreCnn;
      O     #IN_cmd_ShoreBrk_off;
      O     #temp_reset_actProcess;
      )     ;
      R     #stat_c_shore_on;
      U     #stat_c_shore_on;
      )     ;
      =     #OUT_e_stpDieselMan;
NETWORK
TITLE =[6]DG->Shore -Open SC_Breaker in case of a running generator
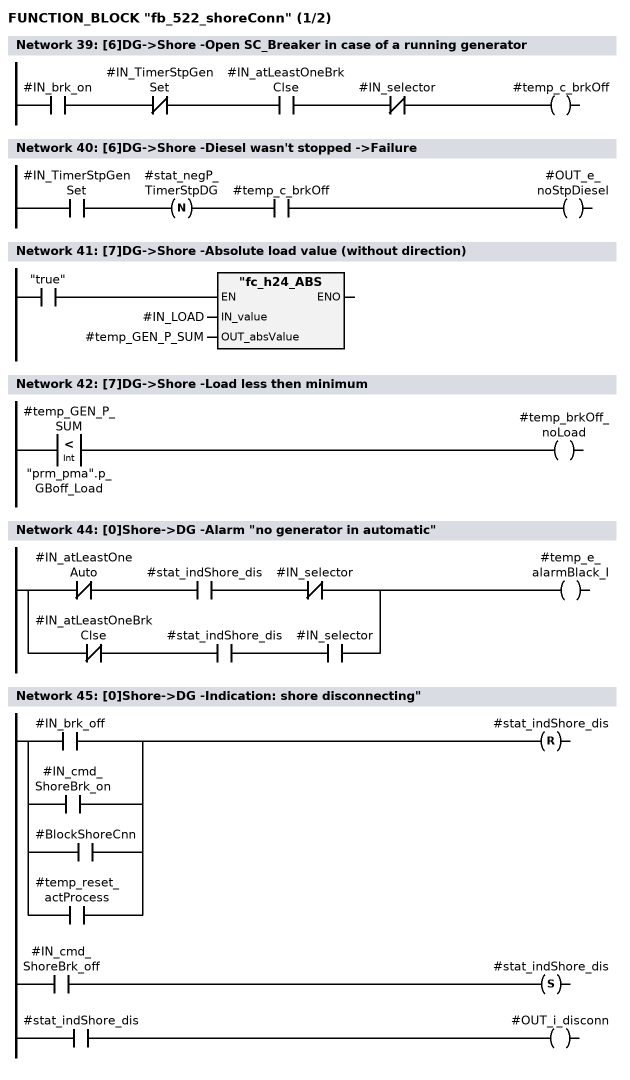
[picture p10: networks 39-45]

      U     #IN_brk_on;
      UN    #IN_TimerStpGenSet;
      U     #IN_atLeastOneBrkClse;
      UN    #IN_selector;
      =     #temp_c_brkOff;
NETWORK
TITLE =[6]DG->Shore -Diesel wasn't stopped ->Failure

      U     #IN_TimerStpGenSet;
      FN    #stat_negP_TimerStpDG;
      U     #temp_c_brkOff;
      =     #OUT_e_noStpDiesel;
NETWORK
TITLE =[7]DG->Shore -Absolute load value (without direction)

      U     "true";
      SPBNB _031;
      CALL "fc_h24_ABS(INT)" (
           IN_value                 := #IN_LOAD,
           OUT_absValue             := #temp_GEN_P_SUM);
_031: NOP   0;
NETWORK
TITLE =[7]DG->Shore -Load less then minimum

      L     #temp_GEN_P_SUM;
      L     "prm_pma".p_GBoff_Load;
      <I    ;
      =     #temp_brkOff_noLoad;
NETWORK
TITLE =



NETWORK
TITLE =[0]Shore->DG -Alarm "no generator in automatic"

      UN    #IN_atLeastOneAuto;
      U     #stat_indShore_dis;
      UN    #IN_selector;
      O     ;
      UN    #IN_atLeastOneBrkClse;
      U     #stat_indShore_dis;
      U     #IN_selector;
      =     #temp_e_alarmBlack_I;
NETWORK
TITLE =[0]Shore->DG -Indication: shore disconnecting"

      U(    ;
      O     #IN_brk_off;
      O     #IN_cmd_ShoreBrk_on;
      O     #BlockShoreCnn;
      O     #temp_reset_actProcess;
      )     ;
      R     #stat_indShore_dis;
      U     #IN_cmd_ShoreBrk_off;
      S     #stat_indShore_dis;
      U     #stat_indShore_dis;
      =     #OUT_i_disconn;
NETWORK
TITLE =[1]Shore->DG -Adjusting the voltage controller
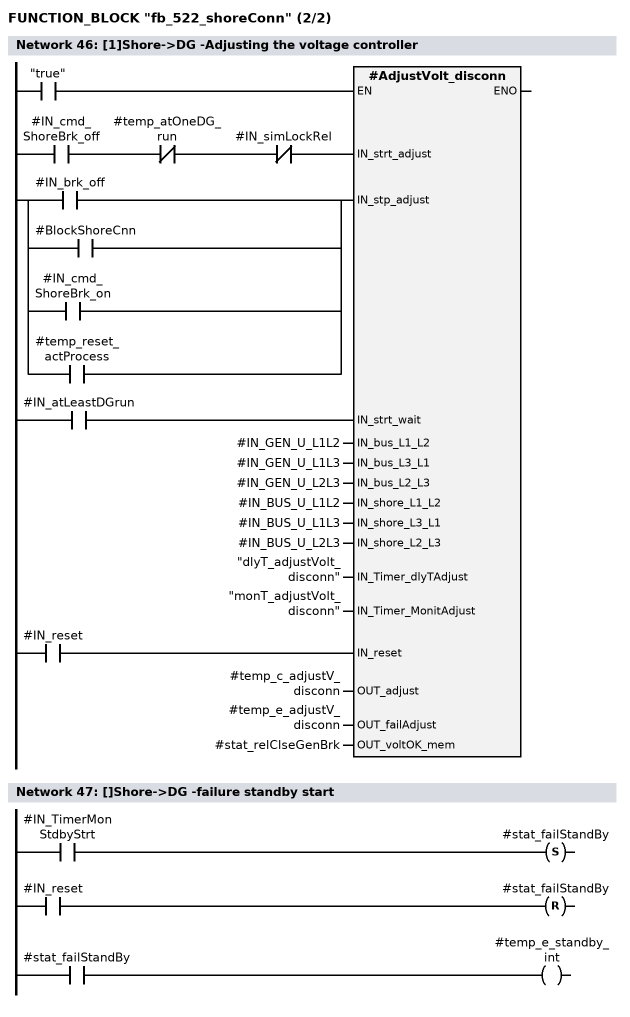
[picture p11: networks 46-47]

      U     #IN_cmd_ShoreBrk_off;
      UN    #temp_atOneDG_run;
      UN    #IN_simLockRel;
      =     L     54.0;
      BLD   103;
      U(    ;
      O     #IN_brk_off;
      O     #BlockShoreCnn;
      O     #IN_cmd_ShoreBrk_on;
      O     #temp_reset_actProcess;
      )     ;
      =     L     54.1;
      BLD   103;
      U     #IN_atLeastDGrun;
      =     L     54.2;
      BLD   103;
      U     #IN_reset;
      =     L     54.3;
      BLD   103;
      U     "true";
      SPBNB _032;
      CALL #AdjustVolt_disconn (
           IN_strt_adjust           := L     54.0,
           IN_stp_adjust            := L     54.1,
           IN_strt_wait             := L     54.2,
           IN_bus_L1_L2             := #IN_GEN_U_L1L2,
           IN_bus_L3_L1             := #IN_GEN_U_L1L3,
           IN_bus_L2_L3             := #IN_GEN_U_L2L3,
           IN_shore_L1_L2           := #IN_BUS_U_L1L2,
           IN_shore_L3_L1           := #IN_BUS_U_L1L3,
           IN_shore_L2_L3           := #IN_BUS_U_L2L3,
           IN_Timer_dlyTAdjust      := "dlyT_adjustVolt_disconn",
           IN_Timer_MonitAdjust     := "monT_adjustVolt_disconn",
           IN_reset                 := L     54.3,
           OUT_adjust               := #temp_c_adjustV_disconn,
           OUT_failAdjust           := #temp_e_adjustV_disconn,
           OUT_voltOK_mem           := #stat_relClseGenBrk);
_032: NOP   0;
NETWORK
TITLE =[]Shore->DG -failure standby start

      U     #IN_TimerMonStdbyStrt;
      S     #stat_failStandBy;
      U     #IN_reset;
      R     #stat_failStandBy;
      U     #stat_failStandBy;
      =     #temp_e_standby_int;
NETWORK
TITLE =[1]Shore->DG -Diesel standby start
//
//
      U     #IN_TimerMonStdbyStrt;
      UN    #IN_cmd_ShoreBrk_off;
      =     L     54.0;
      U(    ;
      O     L     54.0;
      O     #step2_c_brk_off;
      O     #BlockShoreCnn;
      O     #IN_cmd_ShoreBrk_on;
      O     #temp_reset_actProcess;
      )     ;
      R     #step1_c_brk_off;
      U     #IN_cmd_ShoreBrk_off;
      UN    #temp_atOneDG_run;
      UN    #IN_simLockRel;
      S     #step1_c_brk_off;
      U     #step1_c_brk_off;
      L     "prm_pma".p_monT_GenSetOnBus;
      SE    #IN_TimerMonStdbyStrt;
      U     L     54.0;
      BLD   102;
      =     #temp_e_alarmBlack_II;
NETWORK
TITLE =[2]Shore->DG -Failure Diesel take over load
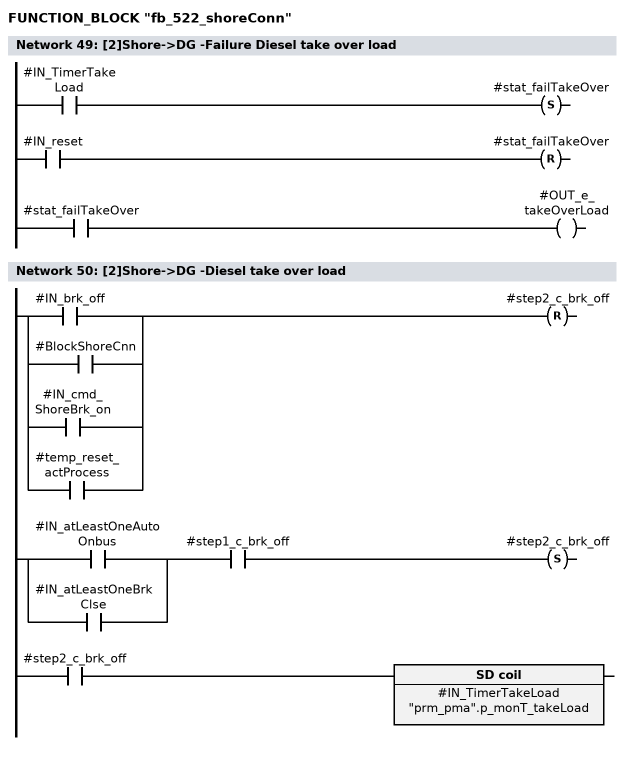
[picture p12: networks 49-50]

      U     #IN_TimerTakeLoad;
      S     #stat_failTakeOver;
      U     #IN_reset;
      R     #stat_failTakeOver;
      U     #stat_failTakeOver;
      =     #OUT_e_takeOverLoad;
NETWORK
TITLE =[2]Shore->DG -Diesel take over load

      U(    ;
      O     #IN_brk_off;
      O     #BlockShoreCnn;
      O     #IN_cmd_ShoreBrk_on;
      O     #temp_reset_actProcess;
      )     ;
      R     #step2_c_brk_off;
      U(    ;
      O     #IN_atLeastOneAutoOnbus;
      O     #IN_atLeastOneBrkClse;
      )     ;
      U     #step1_c_brk_off;
      S     #step2_c_brk_off;
      U     #step2_c_brk_off;
      L     "prm_pma".p_monT_takeLoad;
      SE    #IN_TimerTakeLoad;
NETWORK
TITLE =[2]Shore->DG -Diesel take over load (mode =import)

      U     #IN_atLeastOneAutoOnbus;
      U     #step2_c_brk_off;
      UN    #IN_selector;
      =     L     54.0;
      U     L     54.0;
      BLD   102;
      =     #OUT_c_takeoverLoad;
      O     L     54.0;
      O     ;
      U     #temp_brkOff_noLoad;
      U     #step2_c_brk_off;
      =     #temp_c_brkLoadRed;
NETWORK
TITLE =[2]Shore->DG -Diesel take over load (mode =export)
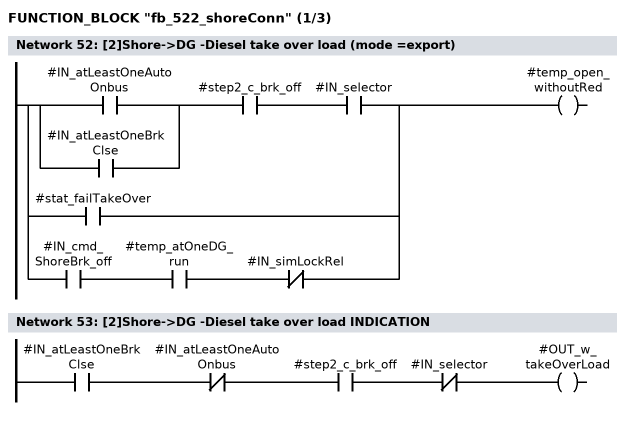
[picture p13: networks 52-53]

      U(    ;
      O     #IN_atLeastOneAutoOnbus;
      O     #IN_atLeastOneBrkClse;
      )     ;
      U     #step2_c_brk_off;
      U     #IN_selector;
      O     #stat_failTakeOver;
      O     ;
      U     #IN_cmd_ShoreBrk_off;
      U     #temp_atOneDG_run;
      UN    #IN_simLockRel;
      =     #temp_open_withoutRed;
NETWORK
TITLE =[2]Shore->DG -Diesel take over load INDICATION

      U     #IN_atLeastOneBrkClse;
      UN    #IN_atLeastOneAutoOnbus;
      U     #step2_c_brk_off;
      UN    #IN_selector;
      =     #OUT_w_takeOverLoad;
NETWORK
TITLE =[2],[4]DG->Shore |[3]Shore->DG -Control SC-breaker (FB51)
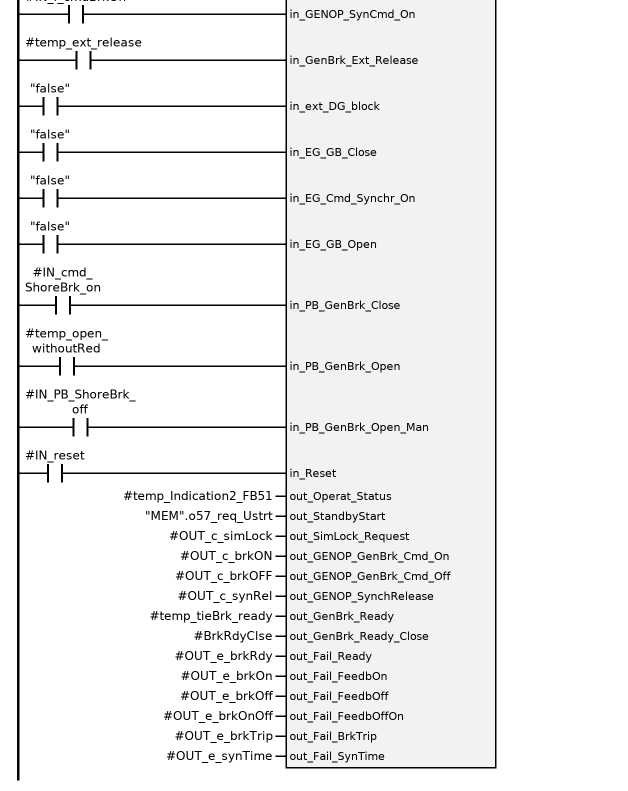
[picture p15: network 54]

      U(    ;
      O     #temp_brkOff_noLoad;
      O     #temp_e_adjustV_disconn;
      )     ;
      =     L     54.0;
      BLD   103;
      U     "false";
      =     L     54.1;
      BLD   103;
      U     #temp_blackout;
      =     L     54.2;
      BLD   103;
      U     #IN_simLock_blc;
      =     L     54.3;
      BLD   103;
      U(    ;
      O     #IN_simLock_err;
      O     #OUT_e_adjustVolt;
      )     ;
      =     L     54.4;
      BLD   103;
      U(    ;
      O     #stat_relSimLock;
      O     #temp_blackout;
      )     ;
      U     #IN_simLockRel;
      =     L     54.5;
      BLD   103;
      U     "true";
      =     L     54.6;
      BLD   103;
      U     "false";
      =     L     54.7;
      BLD   103;
      U(    ;
      O     #temp_c_brkLoadRed;
      O     #temp_c_brkOff;
      )     ;
      =     L     55.0;
      BLD   103;
      U(    ;
      O     #IN_PB_ShoreBrk_off;
      O     #IN_extShoreBrk_openCmd;
      )     ;
      =     L     55.1;
      BLD   103;
      U     #temp_Brk_off;
      =     L     55.2;
      BLD   103;
      U     "false";
      =     L     55.3;
      BLD   103;
      U     "false";
      =     L     55.4;
      BLD   103;
      U     "true";
      =     L     55.5;
      BLD   103;
      U     #IN_brk_ready;
      =     L     55.6;
      BLD   103;
      U     "false";
      =     L     55.7;
      BLD   103;
      U     #IN_brk_normPos;
      UN    #IN_extBlock;
      =     L     56.0;
      BLD   103;
      U     #IN_brk_testPos;
      UN    #IN_extBlock;
      =     L     56.1;
      BLD   103;
      U     #IN_brk_on;
      =     L     56.2;
      BLD   103;
      U     #IN_brk_off;
      =     L     56.3;
      BLD   103;
      U     #IN_f_cmdBrkOn;
      =     L     56.4;
      BLD   103;
      U     #temp_ext_release;
      =     L     56.5;
      BLD   103;
      U     "false";
      =     L     56.6;
      BLD   103;
      U     "false";
      =     L     56.7;
      BLD   103;
      U     "false";
      =     L     57.0;
      BLD   103;
      U     "false";
      =     L     57.1;
      BLD   103;
      U     #IN_cmd_ShoreBrk_on;
      =     L     57.2;
      BLD   103;
      U     #temp_open_withoutRed;
      =     L     57.3;
      BLD   103;
      U     #IN_PB_ShoreBrk_off;
      =     L     57.4;
      BLD   103;
      U     #IN_reset;
      =     L     57.6;
      BLD   103;
      U     "true";
      SPBNB _033;
      CALL #Breaker_control (
           in_DGLoad_off            := L     54.0,
           in_Nmb_Gen_LoadSh        := #temp_No_busbar,
           in_act_mode              := "MEM".o51_mode_bin,
           in_EG_Set                := L     54.1,
           in_Blackout              := L     54.2,
           in_SimLock_Blocked       := L     54.3,
           in_SimLock_Fault         := L     54.4,
           in_SimLock_Release       := L     54.5,
           in_DGWG_run              := L     54.6,
           in_DGWG_Stop             := L     54.7,
           in_GenBrkOff_LoadRed     := L     55.0,
           in_DGWG_GenBrk_Cmd_Off   := L     55.1,
           in_DGWG_GenBrk_Cmd_Trip  := L     55.2,
           in_ChOver_Blackout       := L     55.3,
           in_Standby_ReadyConn     := L     55.4,
           in_ShoreConn_Off         := L     55.5,
           in_DI_GenBrk_ReadyClose  := L     55.6,
           in_DI_GenBrk_Tripped     := L     55.7,
           in_DI_GenBrk_PosNorm     := L     56.0,
           in_DI_GenBrk_PosTest     := L     56.1,
           in_DI_GenBrk_FB_On       := L     56.2,
           in_DI_GenBrk_FB_Off      := L     56.3,
           in_GENOP_SynCmd_On       := L     56.4,
           in_GenBrk_Ext_Release    := L     56.5,
           in_ext_DG_block          := L     56.6,
           in_EG_GB_Close           := L     56.7,
           in_EG_Cmd_Synchr_On      := L     57.0,
           in_EG_GB_Open            := L     57.1,
           in_PB_GenBrk_Close       := L     57.2,
           in_PB_GenBrk_Open        := L     57.3,
           in_PB_GenBrk_Open_Man    := L     57.4,
           in_Reset                 := L     57.6,
           out_Operat_Status        := #temp_Indication2_FB51,
           out_StandbyStart         := "MEM".o57_req_Ustrt,
           out_SimLock_Request      := #OUT_c_simLock,
           out_GENOP_GenBrk_Cmd_On  := #OUT_c_brkON,
           out_GENOP_GenBrk_Cmd_Off := #OUT_c_brkOFF,
           out_GENOP_SynchRelease   := #OUT_c_synRel,
           out_GenBrk_Ready         := #temp_tieBrk_ready,
           out_GenBrk_Ready_Close   := #BrkRdyClse,
           out_Fail_Ready           := #OUT_e_brkRdy,
           out_Fail_FeedbOn         := #OUT_e_brkOn,
           out_Fail_FeedbOff        := #OUT_e_brkOff,
           out_Fail_FeedbOffOn      := #OUT_e_brkOnOff,
           out_Fail_BrkTrip         := #OUT_e_brkTrip,
           out_Fail_SynTime         := #OUT_e_synTime);

_033: NOP   0;
NETWORK
TITLE =DG->Shore -lock the controller
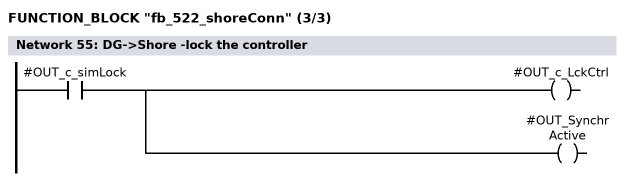
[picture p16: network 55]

      U     #OUT_c_simLock;
      =     #OUT_c_LckCtrl;
      =     #OUT_SynchrActive;
NETWORK
TITLE =POSTCON -command "adjusting voltage"

      O(    ;
      U     #temp_c_adjustV_conn;
      L     "prm_pma".p_dlyT_adj_V_swon;
      SA    "spann_anp_la_einsch";
      NOP   0;
      NOP   0;
      NOP   0;
      U     "spann_anp_la_einsch";
      )     ;
      O(    ;
      U     #temp_c_adjustV_disconn;
      L     "prm_pma".p_dlyT_adj_V_swoff;
      SA    "spann_anp_la_aussch";
      NOP   0;
      NOP   0;
      NOP   0;
      U     "spann_anp_la_aussch";
      )     ;
      =     #OUT_c_adjustVolt;
NETWORK
TITLE =POSTCON -failure "adjusting voltage"
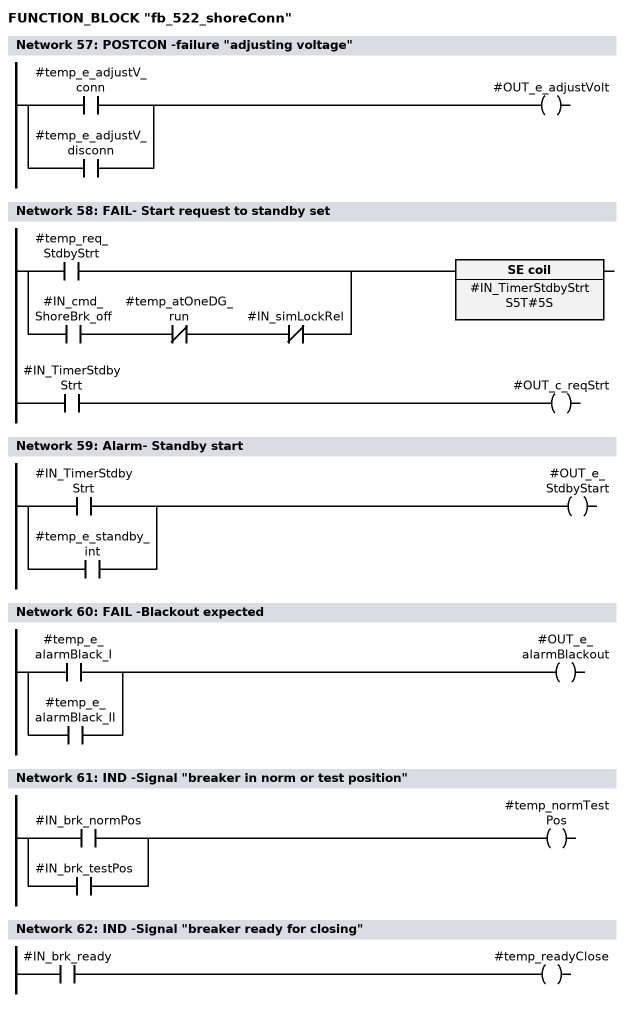
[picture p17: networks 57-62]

      O     #temp_e_adjustV_conn;
      O     #temp_e_adjustV_disconn;
      =     #OUT_e_adjustVolt;
NETWORK
TITLE =FAIL- Start request to standby set

      U(    ;
      O     #temp_req_StdbyStrt;
      O     ;
      U     #IN_cmd_ShoreBrk_off;
      UN    #temp_atOneDG_run;
      UN    #IN_simLockRel;
      )     ;
      L     S5T#5S;
      SV    #IN_TimerStdbyStrt;
      NOP   0;
      NOP   0;
      NOP   0;
      U     #IN_TimerStdbyStrt;
      =     #OUT_c_reqStrt;
NETWORK
TITLE =Alarm- Standby start

      O     #IN_TimerStdbyStrt;
      O     #temp_e_standby_int;
      =     #OUT_e_StdbyStart;
NETWORK
TITLE =FAIL -Blackout expected

      O     #temp_e_alarmBlack_I;
      O     #temp_e_alarmBlack_II;
      =     #OUT_e_alarmBlackout;
NETWORK
TITLE =IND -Signal "breaker in norm or test position"

      O     #IN_brk_normPos;
      O     #IN_brk_testPos;
      =     #temp_normTestPos;
NETWORK
TITLE =IND -Signal "breaker ready for closing"

      U     #IN_brk_ready;
      =     #temp_readyClose;
NETWORK
TITLE =IND -line1:No.47: "shore conn.active, stop diesel"

      L     47;
      U     #IN_brk_on;
      U     #IN_TimerStpGenSet;
      U     #IN_atLeastOneBrkClse;
      SPB   idOP;
NETWORK
TITLE =IND -line1:No.48: "shore conn.finished: start diesel"

      L     48;
      U     #step1_c_brk_off;
      SPB   idOP;
NETWORK
TITLE =IND -line1:No.38: "Tie breaker closed" with kW display

      L     38;
      U     #IN_brk_on;
      SPB   idOP;
NETWORK
TITLE =IND -line1:No.46: "voltage adjusting running"

      L     46;
      U     #OUT_c_adjustVolt;
      UN    #stat_relSimLock;
      SPB   idOP;
NETWORK
TITLE =IND -line1:No.49: "shore conn.finished: take over load"

      L     49;
      U     #step2_c_brk_off;
      SPB   idOP;
NETWORK
TITLE =IND -line1:No.30: "_______" (No indication)
//If there is no indication coming from this FB, "30" is delivered.
      L     30;
idOP: T     #temp_Operat_Status;
NETWORK
TITLE =IND -line 2, no. 1: "press confirmation"

      L     1;
      U     #IN_pressCnfrm;
      SPB   indi;
NETWORK
TITLE =IND -line 2, no. 20: "Blocked"

      L     20;
      U     #BlockShoreCnn;
      SPB   indi;
NETWORK
TITLE =IND -line 2, no. 12: "Tie breaker ready"

      L     12;
      U     #temp_ext_release;
      U     #temp_tieBrk_ready;
      U     #temp_Semi;
      UN    #IN_brk_on;
      UN    #BlockShoreCnn;
      UN    #IN_simLock_err;
      SPB   indi;

NETWORK
TITLE =IND -line 2, no. 11: "Tie breaker not ready"

      L     11;
      U(    ;
      ON    #temp_ext_release;
      ON    #temp_tieBrk_ready;
      ON    #temp_Semi;
      O     #BlockShoreCnn;
      O     #IN_simLock_err;
      )     ;
      UN    #IN_brk_on;
      SPB   indi;
NETWORK
TITLE =IND -line 2, no. 10: "_______" (No indication)
//If there is no indication coming for this line, "10" is delivered.
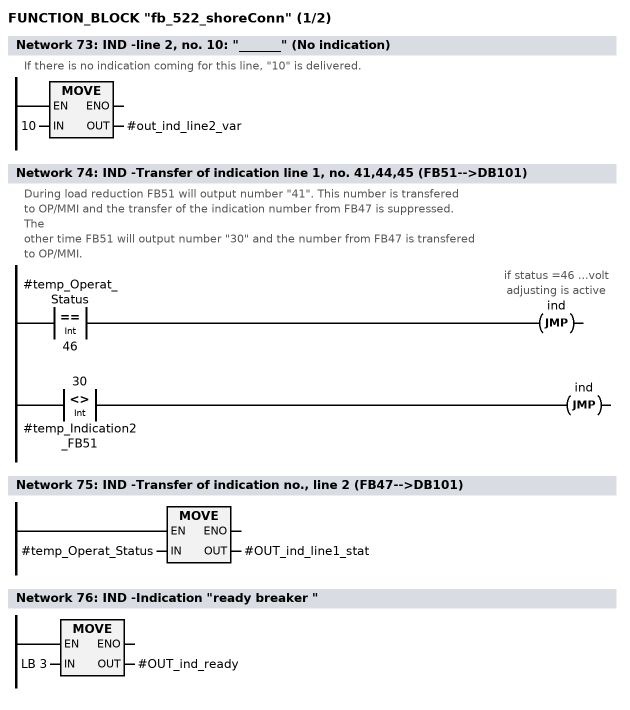
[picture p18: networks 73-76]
      L     10;
indi: T     #out_ind_line2_var;
NETWORK
TITLE =IND -Transfer of indication line 1, no. 41,44,45 (FB51-->DB101)
//During load reduction FB51 will output number "41". This number is transfered
//to OP/MMI and the transfer of the indication number from FB47 is suppressed.
//The
//other time FB51 will output number "30" and the number from FB47 is transfered
//to OP/MMI.
      L     #temp_Operat_Status;
      L     46;
      ==I   ;
      SPB   ind; //if status =46 ...volt adjusting is active

      L     30;
      L     #temp_Indication2_FB51;
      <>I   ;
      SPB   ind;
NETWORK
TITLE =IND -Transfer of indication no., line 2 (FB47-->DB101)

      L     #temp_Operat_Status;
ind:  T     #OUT_ind_line1_stat;
NETWORK
TITLE =IND -Indication "ready breaker "

      L     LB     3;
      T     #OUT_ind_ready;

NETWORK
TITLE =FAIL- Blocking the shore connection breaker
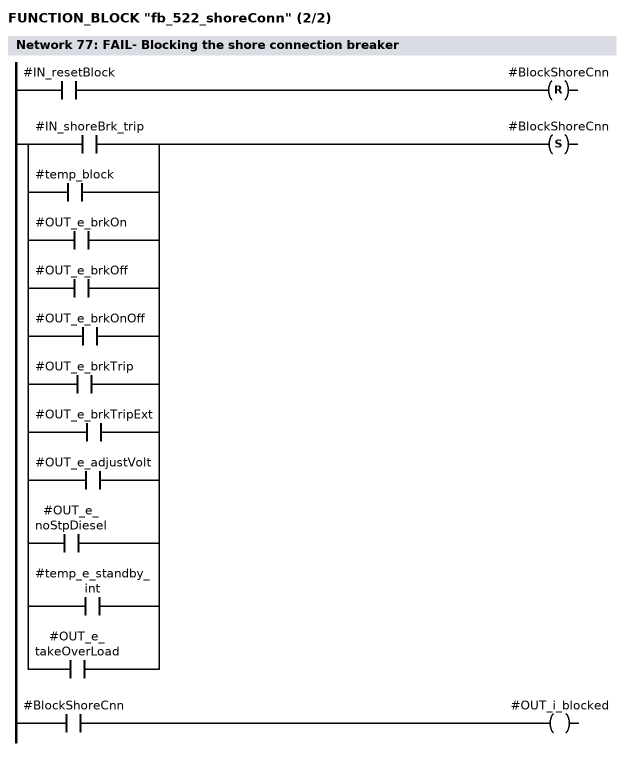
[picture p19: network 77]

      U     #IN_resetBlock;
      R     #BlockShoreCnn;
      U(    ;
      O     #IN_shoreBrk_trip;
      O     #temp_block;
      O     #OUT_e_brkOn;
      O     #OUT_e_brkOff;
      O     #OUT_e_brkOnOff;
      O     #OUT_e_brkTrip;
      O     #OUT_e_brkTripExt;
      O     #OUT_e_adjustVolt;
      O     #OUT_e_noStpDiesel;
      O     #temp_e_standby_int;
      O     #OUT_e_takeOverLoad;
      )     ;
      S     #BlockShoreCnn;
      U     #BlockShoreCnn;
      =     #OUT_i_blocked;
END_FUNCTION_BLOCK

DATA_BLOCK "shore1"
TITLE =
VERSION : 0.0

"fb_522_shoreConn"
BEGIN
   IN_selector := FALSE;
   IN_cmd_ShoreBrk_on := FALSE;
   IN_cmd_ShoreBrk_off := FALSE;
   IN_PB_ShoreBrk_off := FALSE;
   IN_extShoreBrk_openCmd := FALSE;
   IN_extBlock := FALSE;
   IN_blackout_bus := FALSE;
   IN_VoltAvail_bus := FALSE;
   IN_blackout_shore := FALSE;
   IN_shoreVoltAvail := FALSE;
   IN_shortCircuit_otherG := FALSE;
   IN_atLeastOneAuto := FALSE;
   IN_shortCircuit_ext := FALSE;
   IN_atLeastOneAutoOnbus := FALSE;
   IN_atLeastOneBrkClse := FALSE;
   IN_atLeastShoreOn := FALSE;
   IN_atLeastDGrun := FALSE;
   IN_actCfg := W#16#0;
   IN_GEN_I_L1 := 0;
   IN_GEN_I_L2 := 0;
   IN_GEN_I_L3 := 0;
   IN_LOAD := 0;
   IN_BUS_f := 0;
   IN_GEN_f := 0;
   IN_BUS_U_L1L2 := 0;
   IN_BUS_U_L2L3 := 0;
   IN_BUS_U_L1L3 := 0;
   IN_GEN_U_L1L2 := 0;
   IN_GEN_U_L2L3 := 0;
   IN_GEN_U_L1L3 := 0;
   IN_I_SC_GW1 := FALSE;
   IN_I_GW1VER := FALSE;
   IN_I_GW2VER := FALSE;
   IN_I_GW3VER := FALSE;
   IN_I_GW4VER := FALSE;
   IN_P_GW1VER := FALSE;
   IN_simLock_blc := FALSE;
   IN_simLock_err := FALSE;
   IN_simLockRel := FALSE;
   IN_shoreBrk_trip := FALSE;
   IN_brk_ready := FALSE;
   IN_brk_normPos := FALSE;
   IN_brk_testPos := FALSE;
   IN_brk_on := FALSE;
   IN_brk_off := FALSE;
   IN_f_cmdBrkOn := FALSE;
   IN_reset := FALSE;
   IN_resetBlock := FALSE;
   IN_pressCnfrm := FALSE;
   IN_mode := B#16#0;
   IN_TimerStdbyStrt := T 0;
   IN_TimerStpGenSet := T 0;
   IN_TimerStpPulse := T 0;
   IN_TimerMonStdbyStrt := T 0;
   IN_TimerTakeLoad := T 0;
   OUT_SynchrActive := FALSE;
   OUT_c_LckCtrl := FALSE;
   OUT_c_simLock := FALSE;
   OUT_c_brkON := FALSE;
   OUT_c_brkOFF := FALSE;
   OUT_c_synRel := FALSE;
   OUT_c_reqStrt := FALSE;
   OUT_c_reqStp := FALSE;
   OUT_c_adjustVolt := FALSE;
   OUT_c_takeoverLoad := FALSE;
   OUT_c_shortCirc := FALSE;
   OUT_i_blocked := FALSE;
   OUT_i_disconn := FALSE;
   OUT_stdbyNo_1st := B#16#0;
   OUT_e_busbar_monit := FALSE;
   OUT_e_shore_monit := FALSE;
   OUT_e_I_monit := FALSE;
   OUT_e_I := FALSE;
   OUT_e_revP := FALSE;
   OUT_e_I_ov := FALSE;
   OUT_e_P_ov := FALSE;
   OUT_e_f1 := FALSE;
   OUT_e_f2 := FALSE;
   OUT_e_f3 := FALSE;
   OUT_e_f4 := FALSE;
   OUT_e_U1 := FALSE;
   OUT_e_U2 := FALSE;
   OUT_e_U3 := FALSE;
   OUT_e_U4 := FALSE;
   OUT_e_I_sc := FALSE;
   OUT_e_sc_other := FALSE;
   OUT_e_I1 := FALSE;
   OUT_e_I2 := FALSE;
   OUT_e_P1 := FALSE;
   OUT_e_P2 := FALSE;
   OUT_e_black := FALSE;
   OUT_e_brkRdy := FALSE;
   OUT_e_brkOn := FALSE;
   OUT_e_brkOff := FALSE;
   OUT_e_brkOnOff := FALSE;
   OUT_e_brkTrip := FALSE;
   OUT_e_brkTripExt := FALSE;
   OUT_e_synTime := FALSE;
   OUT_e_StdbyStart := FALSE;
   OUT_e_loadTooHigh := FALSE;
   OUT_e_adjustVolt := FALSE;
   OUT_e_warnBlackout := FALSE;
   OUT_e_alarmBlackout := FALSE;
   OUT_e_stpDieselMan := FALSE;
   OUT_e_noStpDiesel := FALSE;
   OUT_e_standByStart := FALSE;
   OUT_e_takeOverLoad := FALSE;
   OUT_w_takeOverLoad := FALSE;
   OUT_ind_ready := B#16#0;
   OUT_ind_line1_stat := 0;
   out_ind_line2_var := 0;
   Gen_Protect.in_GEN_I_L1 := 0;
   Gen_Protect.in_GEN_I_L2 := 0;
   Gen_Protect.in_GEN_I_L3 := 0;
   Gen_Protect.in_GEN_P_SUM := 0;
   Gen_Protect.in_BUS_f := 0;
   Gen_Protect.in_BUS_U_L1L2 := 0;
   Gen_Protect.in_BUS_U_L2L3 := 0;
   Gen_Protect.in_BUS_U_L3L1 := 0;
   Gen_Protect.in_GEN_U_L1L2 := 0;
   Gen_Protect.in_GEN_U_L2L3 := 0;
   Gen_Protect.in_GEN_U_L3L1 := 0;
   Gen_Protect.in_Nmb_Generator := 0;
   Gen_Protect.in_act_mode := B#16#0;
   Gen_Protect.in_EG_Set := FALSE;
   Gen_Protect.in_EG_Harbour_Mode := FALSE;
   Gen_Protect.in_EG_PowerFb_Mode := FALSE;
   Gen_Protect.in_DI_Blackout := FALSE;
   Gen_Protect.in_DI_BusbarVolt := FALSE;
   Gen_Protect.in_DI_FireSpeedRelGenBrk := FALSE;
   Gen_Protect.in_DI_FB_GenBrk_On := FALSE;
   Gen_Protect.in_DI_Wind_Overtemp := FALSE;
   Gen_Protect.in_DiffProt_warn := FALSE;
   Gen_Protect.in_DiffProt_Trip := FALSE;
   Gen_Protect.in_Overc_ShortC_extern := FALSE;
   Gen_Protect.in_GENOP_ShortCircuit := FALSE;
   Gen_Protect.in_GENOP_Overcurrent := FALSE;
   Gen_Protect.in_GENOP_ReversePower := FALSE;
   Gen_Protect.in_GENOP_Unessent1 := FALSE;
   Gen_Protect.in_GENOP_Unessent2 := FALSE;
   Gen_Protect.in_GENOP_Unessent3 := FALSE;
   Gen_Protect.in_Rel_UnderlShd := FALSE;
   Gen_Protect.in_UnderShd_pos := FALSE;
   Gen_Protect.in_ShortCirc_OtherGen := FALSE;
   Gen_Protect.in_Reset := FALSE;
   Gen_Protect.in_p_uncond_reset := FALSE;
   Gen_Protect.out_Blackout := FALSE;
   Gen_Protect.out_BusVolt_avail := FALSE;
   Gen_Protect.out_GenVolt_avail := FALSE;
   Gen_Protect.out_StandbyStart := FALSE;
   Gen_Protect.out_Uness1_Off := FALSE;
   Gen_Protect.out_Uness2_Off := FALSE;
   Gen_Protect.out_Uness3_Off := FALSE;
   Gen_Protect.out_GenBrk_Off := FALSE;
   Gen_Protect.out_ShortCirc_OtherGen := FALSE;
   Gen_Protect.out_VoltContr_Off := FALSE;
   Gen_Protect.out_UndelayStop := FALSE;
   Gen_Protect.out_Blocking := FALSE;
   Gen_Protect.out_ChOver_Semi := FALSE;
   Gen_Protect.out_ChOver_Blackout := FALSE;
   Gen_Protect.out_Underload_Limit := FALSE;
   Gen_Protect.out_Underload_Shd := FALSE;
   Gen_Protect.out_Fail_Busbar := FALSE;
   Gen_Protect.out_Fail_Current := FALSE;
   Gen_Protect.out_Fail_Overcurr := FALSE;
   Gen_Protect.out_Fail_shortCirc := FALSE;
   Gen_Protect.out_Fail_RevPower := FALSE;
   Gen_Protect.out_Fail_overcurrent := FALSE;
   Gen_Protect.out_Fail_overload := FALSE;
   Gen_Protect.out_Fail_Underfrequ1 := FALSE;
   Gen_Protect.out_Fail_Underfrequ2 := FALSE;
   Gen_Protect.out_Fail_Underfrequ3 := FALSE;
   Gen_Protect.out_Fail_Overfrequ := FALSE;
   Gen_Protect.out_Fail_Undervolt1 := FALSE;
   Gen_Protect.out_Fail_Undervolt2 := FALSE;
   Gen_Protect.out_Fail_Overvolt1 := FALSE;
   Gen_Protect.out_Fail_Overvolt2 := FALSE;
   Gen_Protect.out_Fail_ShortCirc_Other := FALSE;
   Gen_Protect.out_Fail_DiffProt_Warn := FALSE;
   Gen_Protect.out_Fail_DiffProt_Trip := FALSE;
   Gen_Protect.out_Fail_Wind_Overtemp := FALSE;
   Gen_Protect.out_Fail_Underload := FALSE;
   Gen_Protect.out_Fail_Underl_SD := FALSE;
   Gen_Protect.out_Spare_1 := FALSE;
   Gen_Protect.out_Spare_2 := FALSE;
   Gen_Protect.out_PrtcEG_sign := DW#16#0;
   Gen_Protect.stat_GEN_I_Min := 0;
   Gen_Protect.stat_GEN_I_Max := 0;
   Gen_Protect.stat_GEN_I_Mean := 0;
   Gen_Protect.stat_BUS_U_Min := 0;
   Gen_Protect.stat_BUS_U_Max := 0;
   Gen_Protect.stat_GEN_U_Min := 0;
   Gen_Protect.stat_GEN_U_Max := 0;
   Gen_Protect.stat_Limit_I1 := FALSE;
   Gen_Protect.stat_Limit_I2 := FALSE;
   Gen_Protect.stat_Limit_I3 := FALSE;
   Gen_Protect.stat_Limit_I4 := FALSE;
   Gen_Protect.stat_Limit_I5 := FALSE;
   Gen_Protect.stat_Limit_I6 := FALSE;
   Gen_Protect.stat_Limit_I7 := FALSE;
   Gen_Protect.stat_Limit_P1 := FALSE;
   Gen_Protect.stat_Limit_P2 := FALSE;
   Gen_Protect.stat_Limit_P3 := FALSE;
   Gen_Protect.stat_Limit_P4 := FALSE;
   Gen_Protect.stat_Limit_P5 := FALSE;
   Gen_Protect.stat_Limit_P6 := FALSE;
   Gen_Protect.stat_Limit_P7 := FALSE;
   Gen_Protect.stat_Limit_f1 := FALSE;
   Gen_Protect.stat_Limit_f2 := FALSE;
   Gen_Protect.stat_Limit_f3 := FALSE;
   Gen_Protect.stat_Limit_f4 := FALSE;
   Gen_Protect.stat_Limit_f5 := FALSE;
   Gen_Protect.stat_Limit_f6 := FALSE;
   Gen_Protect.stat_Limit_f7 := FALSE;
   Gen_Protect.stat_Limit_f8 := FALSE;
   Gen_Protect.stat_Limit_U1 := FALSE;
   Gen_Protect.stat_Limit_U2 := FALSE;
   Gen_Protect.stat_Limit_U3 := FALSE;
   Gen_Protect.stat_Limit_U4 := FALSE;
   Gen_Protect.stat_Limit_P7_undel := FALSE;
   Gen_Protect.stat_Limit_P7_Warn := FALSE;
   Gen_Protect.stat_ShortCircuit := FALSE;
   Gen_Protect.stat_Wind_Overtemp := FALSE;
   Gen_Protect.stat_Standby_ProtWarn := FALSE;
   Gen_Protect.stat_Uness1_TransfLBrk := FALSE;
   Gen_Protect.stat_ShC_OtherSet_Aux := FALSE;
   Gen_Protect.stat_ShC_OtherSet_Pulse := FALSE;
   Gen_Protect.stat_ShC_OtherSet1 := FALSE;
   Gen_Protect.stat_ShC_OtherSet2 := FALSE;
   Gen_Protect.stat_ShC_OtherSet_Reset := FALSE;
   Gen_Protect.stat_Block_ShC_OtherSet := FALSE;
   Gen_Protect.stat_DiffProt_Trip := FALSE;
   Gen_Protect.stat_Trip_Overcurrent := FALSE;
   Gen_Protect.stat_Trip_RevPower := FALSE;
   Gen_Protect.stat_Trip_Underfrequ := FALSE;
   Gen_Protect.stat_Trip_Undervoltage := FALSE;
   Gen_Protect.stat_Uness2_Uness1 := FALSE;
   Gen_Protect.stat_Uness3_Uness2 := FALSE;
   Gen_Protect.stat_GenRunning := FALSE;
   Gen_Protect.stat_Harb_Feedb_Mode := FALSE;
   Gen_Protect.stat_GENOP_StandbySt := FALSE;
   Gen_Protect.stat_FC56_Limit_01 := FALSE;
   Gen_Protect.stat_FC56_Limit_02 := FALSE;
   Gen_Protect.stat_FC56_Limit_03 := FALSE;
   Gen_Protect.stat_FC56_Limit_04 := FALSE;
   Gen_Protect.stat_FC56_Limit_05 := FALSE;
   Gen_Protect.stat_FC56_Limit_06 := FALSE;
   Gen_Protect.stat_FC56_Limit_07 := FALSE;
   Gen_Protect.stat_FC56_Limit_08 := FALSE;
   Gen_Protect.stat_FC56_Limit_09 := FALSE;
   Gen_Protect.stat_FC56_Limit_10 := FALSE;
   Gen_Protect.stat_FC56_Limit_11 := FALSE;
   Gen_Protect.stat_FC56_Limit_12 := FALSE;
   Gen_Protect.stat_FC56_Limit_13 := FALSE;
   Gen_Protect.stat_FC56_Limit_131 := FALSE;
   Gen_Protect.stat_FC56_Limit_14 := FALSE;
   Gen_Protect.stat_FC56_Limit_15 := FALSE;
   Gen_Protect.stat_FC56_Limit_16 := FALSE;
   Gen_Protect.stat_FC56_Limit_17 := FALSE;
   Gen_Protect.stat_FC56_Limit_18 := FALSE;
   Gen_Protect.stat_FC56_Limit_19 := FALSE;
   Gen_Protect.stat_FC56_Limit_20 := FALSE;
   Gen_Protect.stat_FC56_Limit_21 := FALSE;
   Gen_Protect.stat_FC56_Limit_22 := FALSE;
   Gen_Protect.stat_FC56_Limit_23 := FALSE;
   Gen_Protect.stat_FC56_Limit_24 := FALSE;
   Gen_Protect.stat_FC56_Limit_25 := FALSE;
   Gen_Protect.stat_Underload := FALSE;
   Gen_Protect.stat_UndelayStop := FALSE;
   Gen_Protect.stat_Trip_Temp_Overcurr := FALSE;
   Gen_Breaker.in_DGLoad_off := FALSE;
   Gen_Breaker.in_Nmb_Gen_LoadSh := 0;
   Gen_Breaker.in_act_mode := B#16#0;
   Gen_Breaker.in_EG_Set := FALSE;
   Gen_Breaker.in_Blackout := FALSE;
   Gen_Breaker.in_SimLock_Blocked := FALSE;
   Gen_Breaker.in_SimLock_Fault := FALSE;
   Gen_Breaker.in_SimLock_Release := FALSE;
   Gen_Breaker.in_DGWG_run := FALSE;
   Gen_Breaker.in_DGWG_Stop := FALSE;
   Gen_Breaker.in_GenBrkOff_LoadRed := FALSE;
   Gen_Breaker.in_DGWG_GenBrk_Cmd_Off := FALSE;
   Gen_Breaker.in_DGWG_GenBrk_Cmd_Trip := FALSE;
   Gen_Breaker.in_ChOver_Blackout := FALSE;
   Gen_Breaker.in_Standby_ReadyConn := FALSE;
   Gen_Breaker.in_ShoreConn_Off := FALSE;
   Gen_Breaker.in_DI_GenBrk_ReadyClose := FALSE;
   Gen_Breaker.in_DI_GenBrk_Tripped := FALSE;
   Gen_Breaker.in_DI_GenBrk_PosNorm := FALSE;
   Gen_Breaker.in_DI_GenBrk_PosTest := FALSE;
   Gen_Breaker.in_DI_GenBrk_FB_On := FALSE;
   Gen_Breaker.in_DI_GenBrk_FB_Off := FALSE;
   Gen_Breaker.in_GENOP_SynCmd_On := FALSE;
   Gen_Breaker.in_GenBrk_Ext_Release := FALSE;
   Gen_Breaker.in_ext_DG_block := FALSE;
   Gen_Breaker.in_EG_GB_Close := FALSE;
   Gen_Breaker.in_EG_Cmd_Synchr_On := FALSE;
   Gen_Breaker.in_EG_GB_Open := FALSE;
   Gen_Breaker.in_PB_GenBrk_Close := FALSE;
   Gen_Breaker.in_PB_GenBrk_Open := FALSE;
   Gen_Breaker.in_PB_GenBrk_Open_Man := FALSE;
   Gen_Breaker.in_reset_synchron := FALSE;
   Gen_Breaker.in_Reset := FALSE;
   Gen_Breaker.in_power_avail := FALSE;
   Gen_Breaker.out_Operat_Status := 0;
   Gen_Breaker.out_StandbyStart := FALSE;
   Gen_Breaker.out_SimLock_Request := FALSE;
   Gen_Breaker.out_DO_GenBrk_Cmd_Off := FALSE;
   Gen_Breaker.out_GENOP_GenBrk_Cmd_On := FALSE;
   Gen_Breaker.out_GENOP_GenBrk_Cmd_Off := FALSE;
   Gen_Breaker.out_GENOP_SynchRelease := FALSE;
   Gen_Breaker.out_GenBrk_Ready := FALSE;
   Gen_Breaker.out_GenBrk_Ready_Standby := FALSE;
   Gen_Breaker.out_GenBrk_Ready_Close := FALSE;
   Gen_Breaker.out_Brk_Closed_Plausib := FALSE;
   Gen_Breaker.out_UndelayStop := FALSE;
   Gen_Breaker.out_DelayStop := FALSE;
   Gen_Breaker.out_LoadReduction := FALSE;
   Gen_Breaker.out_Blocking := FALSE;
   Gen_Breaker.out_ChOver_Semi := FALSE;
   Gen_Breaker.out_Fail_Ready := FALSE;
   Gen_Breaker.out_Fail_FeedbOn := FALSE;
   Gen_Breaker.out_Fail_FeedbOff := FALSE;
   Gen_Breaker.out_Fail_FeedbOffOn := FALSE;
   Gen_Breaker.out_Fail_BrkTrip := FALSE;
   Gen_Breaker.out_Fail_SynTime := FALSE;
   Gen_Breaker.out_Fail_GenFailure := FALSE;
   Gen_Breaker.out_Fail_ShoreC_GenBrk := FALSE;
   Gen_Breaker.out_Fail_ChgViaBlack := FALSE;
   Gen_Breaker.stat_CntValue01 := 0;
   Gen_Breaker.stat_CntValue02 := 0;
   Gen_Breaker.stat_CntValue03 := 0;
   Gen_Breaker.stat_CntValue04 := 0;
   Gen_Breaker.stat_CntValue05 := 0;
   Gen_Breaker.stat_CntValue06 := 0;
   Gen_Breaker.stat_CntValue07 := 0;
   Gen_Breaker.stat_CntValue08 := 0;
   Gen_Breaker.stat_CntValue09 := 0;
   Gen_Breaker.stat_CntValue10 := 0;
   Gen_Breaker.stat_CntValue11 := 0;
   Gen_Breaker.stat_CntValue12 := 0;
   Gen_Breaker.stat_CntValue13 := 0;
   Gen_Breaker.stat_CntValue14 := 0;
   Gen_Breaker.stat_CntStart01 := FALSE;
   Gen_Breaker.stat_CntStarted01 := FALSE;
   Gen_Breaker.stat_CntStart02 := FALSE;
   Gen_Breaker.stat_CntStarted02 := FALSE;
   Gen_Breaker.stat_CntStart03 := FALSE;
   Gen_Breaker.stat_CntStarted03 := FALSE;
   Gen_Breaker.stat_CntStart04 := FALSE;
   Gen_Breaker.stat_CntStarted04 := FALSE;
   Gen_Breaker.stat_CntStart05 := FALSE;
   Gen_Breaker.stat_CntStarted05 := FALSE;
   Gen_Breaker.stat_CntStart06 := FALSE;
   Gen_Breaker.stat_CntStarted06 := FALSE;
   Gen_Breaker.stat_CntStart07 := FALSE;
   Gen_Breaker.stat_CntStarted07 := FALSE;
   Gen_Breaker.stat_CntStart08 := FALSE;
   Gen_Breaker.stat_CntStarted08 := FALSE;
   Gen_Breaker.stat_CntStart09 := FALSE;
   Gen_Breaker.stat_CntStarted09 := FALSE;
   Gen_Breaker.stat_CntStart10 := FALSE;
   Gen_Breaker.stat_CntStarted10 := FALSE;
   Gen_Breaker.stat_CntStart11 := FALSE;
   Gen_Breaker.stat_CntStarted11 := FALSE;
   Gen_Breaker.stat_CntStart12 := FALSE;
   Gen_Breaker.stat_CntStarted12 := FALSE;
   Gen_Breaker.stat_CntStart13 := FALSE;
   Gen_Breaker.stat_CntStarted13 := FALSE;
   Gen_Breaker.stat_CntStart14 := FALSE;
   Gen_Breaker.stat_CntStarted14 := FALSE;
   Gen_Breaker.stat_BrkReady_TimeEx := FALSE;
   Gen_Breaker.stat_BrkClose_Semi := FALSE;
   Gen_Breaker.stat_BrkOn_Sim := FALSE;
   Gen_Breaker.stat_SynchOn_Pulse := FALSE;
   Gen_Breaker.stat_SynchOn_EG_PAux := FALSE;
   Gen_Breaker.stat_SynchOn := FALSE;
   Gen_Breaker.stat_Synch_TimeEx := FALSE;
   Gen_Breaker.stat_GenBrk_Off_NoLoadR := FALSE;
   Gen_Breaker.stat_GenBrk_Off_LoadRed := FALSE;
   Gen_Breaker.stat_LoadRed_TimeEx := FALSE;
   Gen_Breaker.stat_GenBrkOff_Limit := FALSE;
   Gen_Breaker.stat_GenBrkOff_StbyReady := FALSE;
   Gen_Breaker.stat_FeedbOn_TimeSt := FALSE;
   Gen_Breaker.stat_FeedbOn_TimeEx := FALSE;
   Gen_Breaker.stat_FeedbOff_TimeSt := FALSE;
   Gen_Breaker.stat_FeedbOff_TimeEx := FALSE;
   Gen_Breaker.stat_GenBrk_DelayOff := FALSE;
   Gen_Breaker.stat_PulseAux_Trip := FALSE;
   Gen_Breaker.stat_Fail_GenBrk := FALSE;
   Gen_Breaker.stat_Fail_ShoreC := FALSE;
   Gen_Breaker.stat_synchron := FALSE;
   Gen_Breaker.stat_Fail_GenBrk_TripExt := FALSE;
   Gen_Breaker.stat_PulseAux_GenBrk_Off := FALSE;
   Gen_Breaker.stat_Fail_GenBrk_TripNoR := FALSE;
   Gen_Breaker.stat_GENOP_GenBrk_CmdOff := FALSE;
   Gen_Breaker.stat_power_avail := FALSE;
   Add_Warning.in_PrtcEG_sign := DW#16#0;
   Add_Warning.out_Fail_Warn_Curr_I := FALSE;
   Add_Warning.out_Fail_Warn_Curr_II := FALSE;
   Add_Warning.out_Fail_Warn_Load_I := FALSE;
   Add_Warning.out_Fail_Warn_Load_II := FALSE;
   BlockShoreCnn := FALSE;
   BothSideBlackout := FALSE;
   BrkRdyClse := FALSE;
   Pulse_brk_on := FALSE;
   step1_c_brk_off := FALSE;
   step2_c_brk_off := FALSE;
   stat_relSimLock := FALSE;
   stat_relClseGenBrk := FALSE;
   stat_indShore_dis := FALSE;
   stat_c_shore_on := FALSE;
   stat_negP_TimerStpDG := FALSE;
   stat_failStandBy := FALSE;
   stat_failTakeOver := FALSE;
   stat_failBlackout_SC := FALSE;
   stat_selector_imp := FALSE;
   stat_selector_exp := FALSE;
   Breaker_control.in_DGLoad_off := FALSE;
   Breaker_control.in_Nmb_Gen_LoadSh := 0;
   Breaker_control.in_act_mode := B#16#0;
   Breaker_control.in_EG_Set := FALSE;
   Breaker_control.in_Blackout := FALSE;
   Breaker_control.in_SimLock_Blocked := FALSE;
   Breaker_control.in_SimLock_Fault := FALSE;
   Breaker_control.in_SimLock_Release := FALSE;
   Breaker_control.in_DGWG_run := FALSE;
   Breaker_control.in_DGWG_Stop := FALSE;
   Breaker_control.in_GenBrkOff_LoadRed := FALSE;
   Breaker_control.in_DGWG_GenBrk_Cmd_Off := FALSE;
   Breaker_control.in_DGWG_GenBrk_Cmd_Trip := FALSE;
   Breaker_control.in_ChOver_Blackout := FALSE;
   Breaker_control.in_Standby_ReadyConn := FALSE;
   Breaker_control.in_ShoreConn_Off := FALSE;
   Breaker_control.in_DI_GenBrk_ReadyClose := FALSE;
   Breaker_control.in_DI_GenBrk_Tripped := FALSE;
   Breaker_control.in_DI_GenBrk_PosNorm := FALSE;
   Breaker_control.in_DI_GenBrk_PosTest := FALSE;
   Breaker_control.in_DI_GenBrk_FB_On := FALSE;
   Breaker_control.in_DI_GenBrk_FB_Off := FALSE;
   Breaker_control.in_GENOP_SynCmd_On := FALSE;
   Breaker_control.in_GenBrk_Ext_Release := FALSE;
   Breaker_control.in_ext_DG_block := FALSE;
   Breaker_control.in_EG_GB_Close := FALSE;
   Breaker_control.in_EG_Cmd_Synchr_On := FALSE;
   Breaker_control.in_EG_GB_Open := FALSE;
   Breaker_control.in_PB_GenBrk_Close := FALSE;
   Breaker_control.in_PB_GenBrk_Open := FALSE;
   Breaker_control.in_PB_GenBrk_Open_Man := FALSE;
   Breaker_control.in_reset_synchron := FALSE;
   Breaker_control.in_Reset := FALSE;
   Breaker_control.in_power_avail := FALSE;
   Breaker_control.out_Operat_Status := 0;
   Breaker_control.out_StandbyStart := FALSE;
   Breaker_control.out_SimLock_Request := FALSE;
   Breaker_control.out_DO_GenBrk_Cmd_Off := FALSE;
   Breaker_control.out_GENOP_GenBrk_Cmd_On := FALSE;
   Breaker_control.out_GENOP_GenBrk_Cmd_Off := FALSE;
   Breaker_control.out_GENOP_SynchRelease := FALSE;
   Breaker_control.out_GenBrk_Ready := FALSE;
   Breaker_control.out_GenBrk_Ready_Standby := FALSE;
   Breaker_control.out_GenBrk_Ready_Close := FALSE;
   Breaker_control.out_Brk_Closed_Plausib := FALSE;
   Breaker_control.out_UndelayStop := FALSE;
   Breaker_control.out_DelayStop := FALSE;
   Breaker_control.out_LoadReduction := FALSE;
   Breaker_control.out_Blocking := FALSE;
   Breaker_control.out_ChOver_Semi := FALSE;
   Breaker_control.out_Fail_Ready := FALSE;
   Breaker_control.out_Fail_FeedbOn := FALSE;
   Breaker_control.out_Fail_FeedbOff := FALSE;
   Breaker_control.out_Fail_FeedbOffOn := FALSE;
   Breaker_control.out_Fail_BrkTrip := FALSE;
   Breaker_control.out_Fail_SynTime := FALSE;
   Breaker_control.out_Fail_GenFailure := FALSE;
   Breaker_control.out_Fail_ShoreC_GenBrk := FALSE;
   Breaker_control.out_Fail_ChgViaBlack := FALSE;
   Breaker_control.stat_CntValue01 := 0;
   Breaker_control.stat_CntValue02 := 0;
   Breaker_control.stat_CntValue03 := 0;
   Breaker_control.stat_CntValue04 := 0;
   Breaker_control.stat_CntValue05 := 0;
   Breaker_control.stat_CntValue06 := 0;
   Breaker_control.stat_CntValue07 := 0;
   Breaker_control.stat_CntValue08 := 0;
   Breaker_control.stat_CntValue09 := 0;
   Breaker_control.stat_CntValue10 := 0;
   Breaker_control.stat_CntValue11 := 0;
   Breaker_control.stat_CntValue12 := 0;
   Breaker_control.stat_CntValue13 := 0;
   Breaker_control.stat_CntValue14 := 0;
   Breaker_control.stat_CntStart01 := FALSE;
   Breaker_control.stat_CntStarted01 := FALSE;
   Breaker_control.stat_CntStart02 := FALSE;
   Breaker_control.stat_CntStarted02 := FALSE;
   Breaker_control.stat_CntStart03 := FALSE;
   Breaker_control.stat_CntStarted03 := FALSE;
   Breaker_control.stat_CntStart04 := FALSE;
   Breaker_control.stat_CntStarted04 := FALSE;
   Breaker_control.stat_CntStart05 := FALSE;
   Breaker_control.stat_CntStarted05 := FALSE;
   Breaker_control.stat_CntStart06 := FALSE;
   Breaker_control.stat_CntStarted06 := FALSE;
   Breaker_control.stat_CntStart07 := FALSE;
   Breaker_control.stat_CntStarted07 := FALSE;
   Breaker_control.stat_CntStart08 := FALSE;
   Breaker_control.stat_CntStarted08 := FALSE;
   Breaker_control.stat_CntStart09 := FALSE;
   Breaker_control.stat_CntStarted09 := FALSE;
   Breaker_control.stat_CntStart10 := FALSE;
   Breaker_control.stat_CntStarted10 := FALSE;
   Breaker_control.stat_CntStart11 := FALSE;
   Breaker_control.stat_CntStarted11 := FALSE;
   Breaker_control.stat_CntStart12 := FALSE;
   Breaker_control.stat_CntStarted12 := FALSE;
   Breaker_control.stat_CntStart13 := FALSE;
   Breaker_control.stat_CntStarted13 := FALSE;
   Breaker_control.stat_CntStart14 := FALSE;
   Breaker_control.stat_CntStarted14 := FALSE;
   Breaker_control.stat_BrkReady_TimeEx := FALSE;
   Breaker_control.stat_BrkClose_Semi := FALSE;
   Breaker_control.stat_BrkOn_Sim := FALSE;
   Breaker_control.stat_SynchOn_Pulse := FALSE;
   Breaker_control.stat_SynchOn_EG_PAux := FALSE;
   Breaker_control.stat_SynchOn := FALSE;
   Breaker_control.stat_Synch_TimeEx := FALSE;
   Breaker_control.stat_GenBrk_Off_NoLoadR := FALSE;
   Breaker_control.stat_GenBrk_Off_LoadRed := FALSE;
   Breaker_control.stat_LoadRed_TimeEx := FALSE;
   Breaker_control.stat_GenBrkOff_Limit := FALSE;
   Breaker_control.stat_GenBrkOff_StbyReady := FALSE;
   Breaker_control.stat_FeedbOn_TimeSt := FALSE;
   Breaker_control.stat_FeedbOn_TimeEx := FALSE;
   Breaker_control.stat_FeedbOff_TimeSt := FALSE;
   Breaker_control.stat_FeedbOff_TimeEx := FALSE;
   Breaker_control.stat_GenBrk_DelayOff := FALSE;
   Breaker_control.stat_PulseAux_Trip := FALSE;
   Breaker_control.stat_Fail_GenBrk := FALSE;
   Breaker_control.stat_Fail_ShoreC := FALSE;
   Breaker_control.stat_synchron := FALSE;
   Breaker_control.stat_Fail_GenBrk_TripExt := FALSE;
   Breaker_control.stat_PulseAux_GenBrk_Off := FALSE;
   Breaker_control.stat_Fail_GenBrk_TripNoR := FALSE;
   Breaker_control.stat_GENOP_GenBrk_CmdOff := FALSE;
   Breaker_control.stat_power_avail := FALSE;
   AdjustVolt_conn.IN_strt_adjust := FALSE;
   AdjustVolt_conn.IN_stp_adjust := FALSE;
   AdjustVolt_conn.IN_strt_wait := FALSE;
   AdjustVolt_conn.IN_bus_L1_L2 := 0;
   AdjustVolt_conn.IN_bus_L3_L1 := 0;
   AdjustVolt_conn.IN_bus_L2_L3 := 0;
   AdjustVolt_conn.IN_shore_L1_L2 := 0;
   AdjustVolt_conn.IN_shore_L3_L1 := 0;
   AdjustVolt_conn.IN_shore_L2_L3 := 0;
   AdjustVolt_conn.IN_Timer_dlyTAdjust := T 0;
   AdjustVolt_conn.IN_Timer_MonitAdjust := T 0;
   AdjustVolt_conn.IN_reset := FALSE;
   AdjustVolt_conn.OUT_adjust := FALSE;
   AdjustVolt_conn.OUT_failAdjust := FALSE;
   AdjustVolt_conn.OUT_voltOK_mem := FALSE;
   AdjustVolt_conn.stat_adjustActive := FALSE;
   AdjustVolt_conn.stat_waitTAdjust := FALSE;
   AdjustVolt_conn.stat_adjustFail := FALSE;
   AdjustVolt_disconn.IN_strt_adjust := FALSE;
   AdjustVolt_disconn.IN_stp_adjust := FALSE;
   AdjustVolt_disconn.IN_strt_wait := FALSE;
   AdjustVolt_disconn.IN_bus_L1_L2 := 0;
   AdjustVolt_disconn.IN_bus_L3_L1 := 0;
   AdjustVolt_disconn.IN_bus_L2_L3 := 0;
   AdjustVolt_disconn.IN_shore_L1_L2 := 0;
   AdjustVolt_disconn.IN_shore_L3_L1 := 0;
   AdjustVolt_disconn.IN_shore_L2_L3 := 0;
   AdjustVolt_disconn.IN_Timer_dlyTAdjust := T 0;
   AdjustVolt_disconn.IN_Timer_MonitAdjust := T 0;
   AdjustVolt_disconn.IN_reset := FALSE;
   AdjustVolt_disconn.OUT_adjust := FALSE;
   AdjustVolt_disconn.OUT_failAdjust := FALSE;
   AdjustVolt_disconn.OUT_voltOK_mem := FALSE;
   AdjustVolt_disconn.stat_adjustActive := FALSE;
   AdjustVolt_disconn.stat_waitTAdjust := FALSE;
   AdjustVolt_disconn.stat_adjustFail := FALSE;
END_DATA_BLOCK

FUNCTION "fc_ShoreConn" : VOID
TITLE =Shore connection -one breaker-
//version!date    !author !change_segm!change_description
//-------+--------+-------+-----------+-------------------------------
// 1.0   !17.03.00!Kahle  ! ---       ! 1st version
// 1.1   !27.04.00!Kahle  ! 2         ! new parameter "at least one shore on"
// 1.2   !14.05.01!Kahle  ! 1         ! add.signals"IN_extShoreBrk_OpenCmd",
//       !        !       !           !            "IN_extBlock"
//       !        !       !           ! add.ind."OUT_e_I_ov" & "OUT_e_P_ov"
//       !        !       !           ! del. log.conn "M 97.5"
AUTHOR : Kahle
FAMILY : PMA71
NAME : OneShore
VERSION : 1.2

BEGIN
NETWORK
TITLE =Shore connection breaker 1
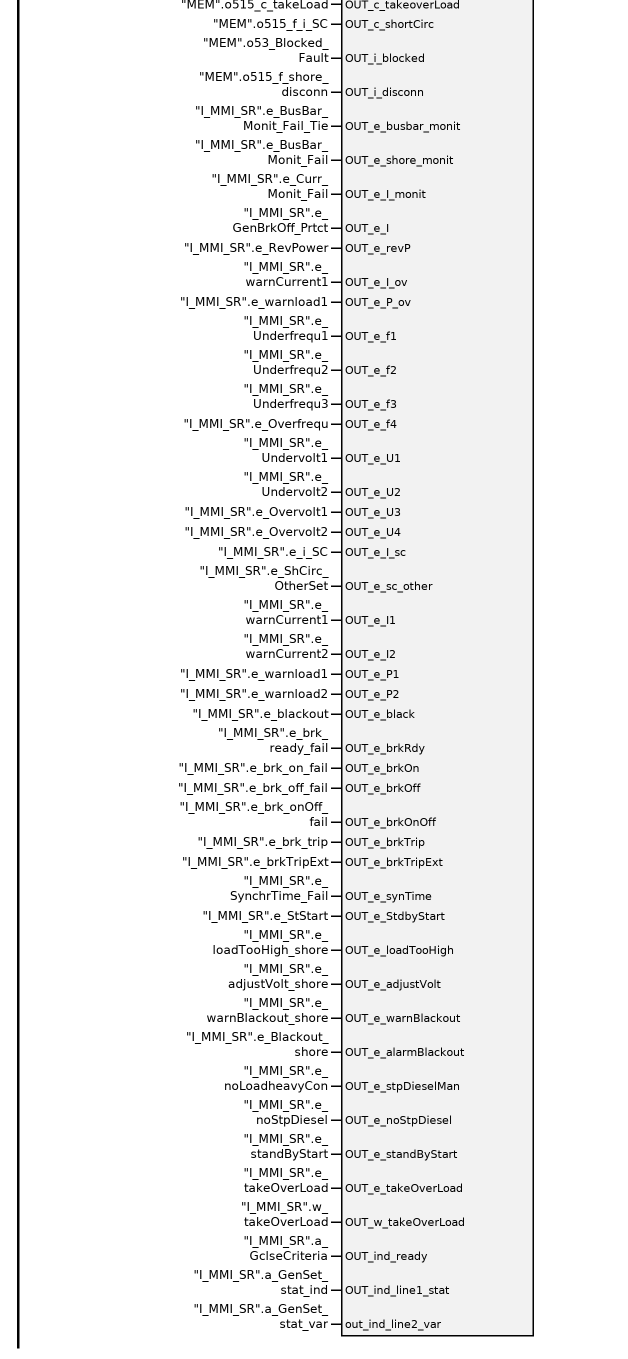
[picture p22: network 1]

      UN    "IN_selector";
      =     L      0.0;
      BLD   103;
      U     "I_MMI_SR".c_genBrk_clse;
      =     L      0.1;
      BLD   103;
      U     "I_MMI_SR".c_genBrk_opn;
      =     L      0.2;
      BLD   103;
      UN    "IN_PB_GenBrk_Off";
      =     L      0.3;
      BLD   103;
      U     "MEM".o57_ExtCBopenCmd;
      =     L      0.4;
      BLD   103;
      U     "MEM".o57_extBlock;
      =     L      0.5;
      BLD   103;
      U     "IN_black_1";
      =     L      0.6;
      BLD   103;
      U     "IN_non_black_2";
      =     L      0.7;
      BLD   103;
      U     "IN_black_shore";
      =     L      1.0;
      BLD   103;
      U     "IN_non_black_shore";
      =     L      1.1;
      BLD   103;
      U     "MEM".o515R_f_i_SC;
      =     L      1.2;
      BLD   103;
      U     "MEM".o515R_f_auto;
      =     L      1.3;
      BLD   103;
      U     "IN_Brk_Tripped";
      =     L      1.4;
      BLD   103;
      U     "MEM".o515R_f_onbus;
      =     L      1.5;
      BLD   103;
      U     "MEM".o515R_f_brk_clse;
      =     L      1.6;
      BLD   103;
      U     "MEM".o515R_f_shoreMode;
      =     L      1.7;
      BLD   103;
      U     "MEM".o515R_f_run;
      =     L      2.0;
      BLD   103;
      U     "I_prtcSR".e_I_SC_VER;
      =     L      2.1;
      BLD   103;
      U     "I_prtcSR".e_I_GW1VER;
      =     L      2.2;
      BLD   103;
      U     "I_prtcSR".e_I_GW2VER;
      =     L      2.3;
      BLD   103;
      U     "I_prtcSR".e_I_GW3VER;
      =     L      2.4;
      BLD   103;
      U     "I_prtcSR".e_I_GW4VER;
      =     L      2.5;
      BLD   103;
      U     "I_prtcSR".e_P_GW1VER;
      =     L      2.6;
      BLD   103;
      U     "MEM".o515_ownBlock;
      =     L      2.7;
      BLD   103;
      U     "MEM".o515_simulLockErr;
      =     L      3.0;
      BLD   103;
      U     "MEM".o515_simulLockAct;
      =     L      3.1;
      BLD   103;
      U     "IN_brk_prepared";
      =     L      3.3;
      BLD   103;
      U     "IN_brk_normPos";
      =     L      3.4;
      BLD   103;
      U     "IN_brk_testPos";
      =     L      3.5;
      BLD   103;
      U     "IN_brk_clse";
      =     L      3.6;
      BLD   103;
      U     "IN_brk_opn";
      =     L      3.7;
      BLD   103;
      U     "I_prtcSR".i_BR_ON;
      =     L      4.0;
      BLD   103;
      U     "I_MMI_SR".c_rst_alm;
      =     L      4.1;
      BLD   103;
      U     "MEM".o51_blockF_reset;
      =     L      4.2;
      BLD   103;
      U     "MEM".o51_i_pressCnfrm;
      =     L      4.3;
      BLD   103;
      U(    ;
      O     "IN_shoreBrk1_trip";
      O     "IN_shoreBrk2_trip";
      O     "IN_shoreBrk3_trip";
      O     "IN_shoreBrk4_trip";
      )     ;
      SPBNB _001;
      CALL "fb_522_shoreConn" , "shore1" (
           IN_selector              := L      0.0,
           IN_cmd_ShoreBrk_on       := L      0.1,
           IN_cmd_ShoreBrk_off      := L      0.2,
           IN_PB_ShoreBrk_off       := L      0.3,
           IN_extShoreBrk_openCmd   := L      0.4,
           IN_extBlock              := L      0.5,
           IN_blackout_bus          := L      0.6,
           IN_VoltAvail_bus         := L      0.7,
           IN_blackout_shore        := L      1.0,
           IN_shoreVoltAvail        := L      1.1,
           IN_shortCircuit_otherG   := L      1.2,
           IN_atLeastOneAuto        := L      1.3,
           IN_shortCircuit_ext      := L      1.4,
           IN_atLeastOneAutoOnbus   := L      1.5,
           IN_atLeastOneBrkClse     := L      1.6,
           IN_atLeastShoreOn        := L      1.7,
           IN_atLeastDGrun          := L      2.0,
           IN_actCfg                := "MEM".o51_actCfg,
           IN_GEN_I_L1              := "I_prtcSR".a_I_L1,
           IN_GEN_I_L2              := "I_prtcSR".a_I_L2,
           IN_GEN_I_L3              := "I_prtcSR".a_I_L3,
           IN_LOAD                  := "I_prtcSR".a_P_SUM,
           IN_BUS_f                 := "I_prtcSR".a_FREQ_BUS,
           IN_GEN_f                 := "I_prtcSR".a_FREQ_GEN,
           IN_BUS_U_L1L2            := "I_prtcSR".a_BUS_L1_L2,
           IN_BUS_U_L2L3            := "I_prtcSR".a_BUS_L2_L3,
           IN_BUS_U_L1L3            := "I_prtcSR".a_BUS_L1_L3,
           IN_GEN_U_L1L2            := "I_prtcSR".a_GEN_L1_L2,
           IN_GEN_U_L2L3            := "I_prtcSR".a_GEN_L2_L3,
           IN_GEN_U_L1L3            := "I_prtcSR".a_GEN_L1_L3,
           IN_I_SC_GW1              := L      2.1,
           IN_I_GW1VER              := L      2.2,
           IN_I_GW2VER              := L      2.3,
           IN_I_GW3VER              := L      2.4,
           IN_I_GW4VER              := L      2.5,
           IN_P_GW1VER              := L      2.6,
           IN_simLock_blc           := L      2.7,
           IN_simLock_err           := L      3.0,
           IN_simLockRel            := L      3.1,
           IN_brk_ready             := L      3.3,
           IN_brk_normPos           := L      3.4,
           IN_brk_testPos           := L      3.5,
           IN_brk_on                := L      3.6,
           IN_brk_off               := L      3.7,
           IN_f_cmdBrkOn            := L      4.0,
           IN_reset                 := L      4.1,
           IN_resetBlock            := L      4.2,
           IN_pressCnfrm            := L      4.3,
           IN_mode                  := "MEM".o51_mode_bin,
           IN_TimerStdbyStrt        := "dlyT_StdByStrt_shore",
           IN_TimerStpGenSet        := "monT_StpGen_shore",
           IN_TimerStpPulse         := "dlyT_adjustVolt_conn",
           IN_TimerMonStdbyStrt     := "monT_StdByStrt_shore",
           IN_TimerTakeLoad         := "monT_TakeLoad_shore",
           OUT_SynchrActive         := "OUT_synchrActive",
           OUT_c_LckCtrl            := "MEM".o515_c_LckCtrl,
           OUT_c_simLock            := "MEM".o515_c_simulLock,
           OUT_c_brkON              := "I_prtcSR".c_BR_ON,
           OUT_c_brkOFF             := "I_prtcSR".c_BR_OFF,
           OUT_c_synRel             := "I_prtcSR".c_SYN_EN,
           OUT_c_reqStrt            := "MEM".o515_c_reqStrt,
           OUT_c_reqStp             := "MEM".o515_c_shoreOn,
           OUT_c_adjustVolt         := "OUT_adjustVolt",
           OUT_c_takeoverLoad       := "MEM".o515_c_takeLoad,
           OUT_c_shortCirc          := "MEM".o515_f_i_SC,
           OUT_i_blocked            := "MEM".o53_Blocked_Fault,
           OUT_i_disconn            := "MEM".o515_f_shore_disconn,
           OUT_e_busbar_monit       := "I_MMI_SR".e_BusBar_Monit_Fail_Tie,
           OUT_e_shore_monit        := "I_MMI_SR".e_BusBar_Monit_Fail,
           OUT_e_I_monit            := "I_MMI_SR".e_Curr_Monit_Fail,
           OUT_e_I                  := "I_MMI_SR".e_GenBrkOff_Prtct,
           OUT_e_revP               := "I_MMI_SR".e_RevPower,
           OUT_e_I_ov               := "I_MMI_SR".e_warnCurrent1,
           OUT_e_P_ov               := "I_MMI_SR".e_warnload1,
           OUT_e_f1                 := "I_MMI_SR".e_Underfrequ1,
           OUT_e_f2                 := "I_MMI_SR".e_Underfrequ2,
           OUT_e_f3                 := "I_MMI_SR".e_Underfrequ3,
           OUT_e_f4                 := "I_MMI_SR".e_Overfrequ,
           OUT_e_U1                 := "I_MMI_SR".e_Undervolt1,
           OUT_e_U2                 := "I_MMI_SR".e_Undervolt2,
           OUT_e_U3                 := "I_MMI_SR".e_Overvolt1,
           OUT_e_U4                 := "I_MMI_SR".e_Overvolt2,
           OUT_e_I_sc               := "I_MMI_SR".e_i_SC,
           OUT_e_sc_other           := "I_MMI_SR".e_ShCirc_OtherSet,
           OUT_e_I1                 := "I_MMI_SR".e_warnCurrent1,
           OUT_e_I2                 := "I_MMI_SR".e_warnCurrent2,
           OUT_e_P1                 := "I_MMI_SR".e_warnload1,
           OUT_e_P2                 := "I_MMI_SR".e_warnload2,
           OUT_e_black              := "I_MMI_SR".e_blackout,
           OUT_e_brkRdy             := "I_MMI_SR".e_brk_ready_fail,
           OUT_e_brkOn              := "I_MMI_SR".e_brk_on_fail,
           OUT_e_brkOff             := "I_MMI_SR".e_brk_off_fail,
           OUT_e_brkOnOff           := "I_MMI_SR".e_brk_onOff_fail,
           OUT_e_brkTrip            := "I_MMI_SR".e_brk_trip,
           OUT_e_brkTripExt         := "I_MMI_SR".e_brkTripExt,
           OUT_e_synTime            := "I_MMI_SR".e_SynchrTime_Fail,
           OUT_e_StdbyStart         := "I_MMI_SR".e_StStart,
           OUT_e_loadTooHigh        := "I_MMI_SR".e_loadTooHigh_shore,
           OUT_e_adjustVolt         := "I_MMI_SR".e_adjustVolt_shore,
           OUT_e_warnBlackout       := "I_MMI_SR".e_warnBlackout_shore,
           OUT_e_alarmBlackout      := "I_MMI_SR".e_Blackout_shore,
           OUT_e_stpDieselMan       := "I_MMI_SR".e_noLoadheavyCon,
           OUT_e_noStpDiesel        := "I_MMI_SR".e_noStpDiesel,
           OUT_e_standByStart       := "I_MMI_SR".e_standByStart,
           OUT_e_takeOverLoad       := "I_MMI_SR".e_takeOverLoad,
           OUT_w_takeOverLoad       := "I_MMI_SR".w_takeOverLoad,
           OUT_ind_ready            := "I_MMI_SR".a_GclseCriteria,
           OUT_ind_line1_stat       := "I_MMI_SR".a_GenSet_stat_ind,
           out_ind_line2_var        := "I_MMI_SR".a_GenSet_stat_var);
_001: NOP   0;
NETWORK
TITLE =To MMI: Failure of simultaneous locking (time exceeded)
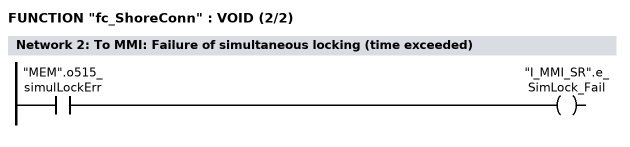
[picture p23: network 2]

      U     "MEM".o515_simulLockErr;
      =     "I_MMI_SR".e_SimLock_Fail;
END_FUNCTION

